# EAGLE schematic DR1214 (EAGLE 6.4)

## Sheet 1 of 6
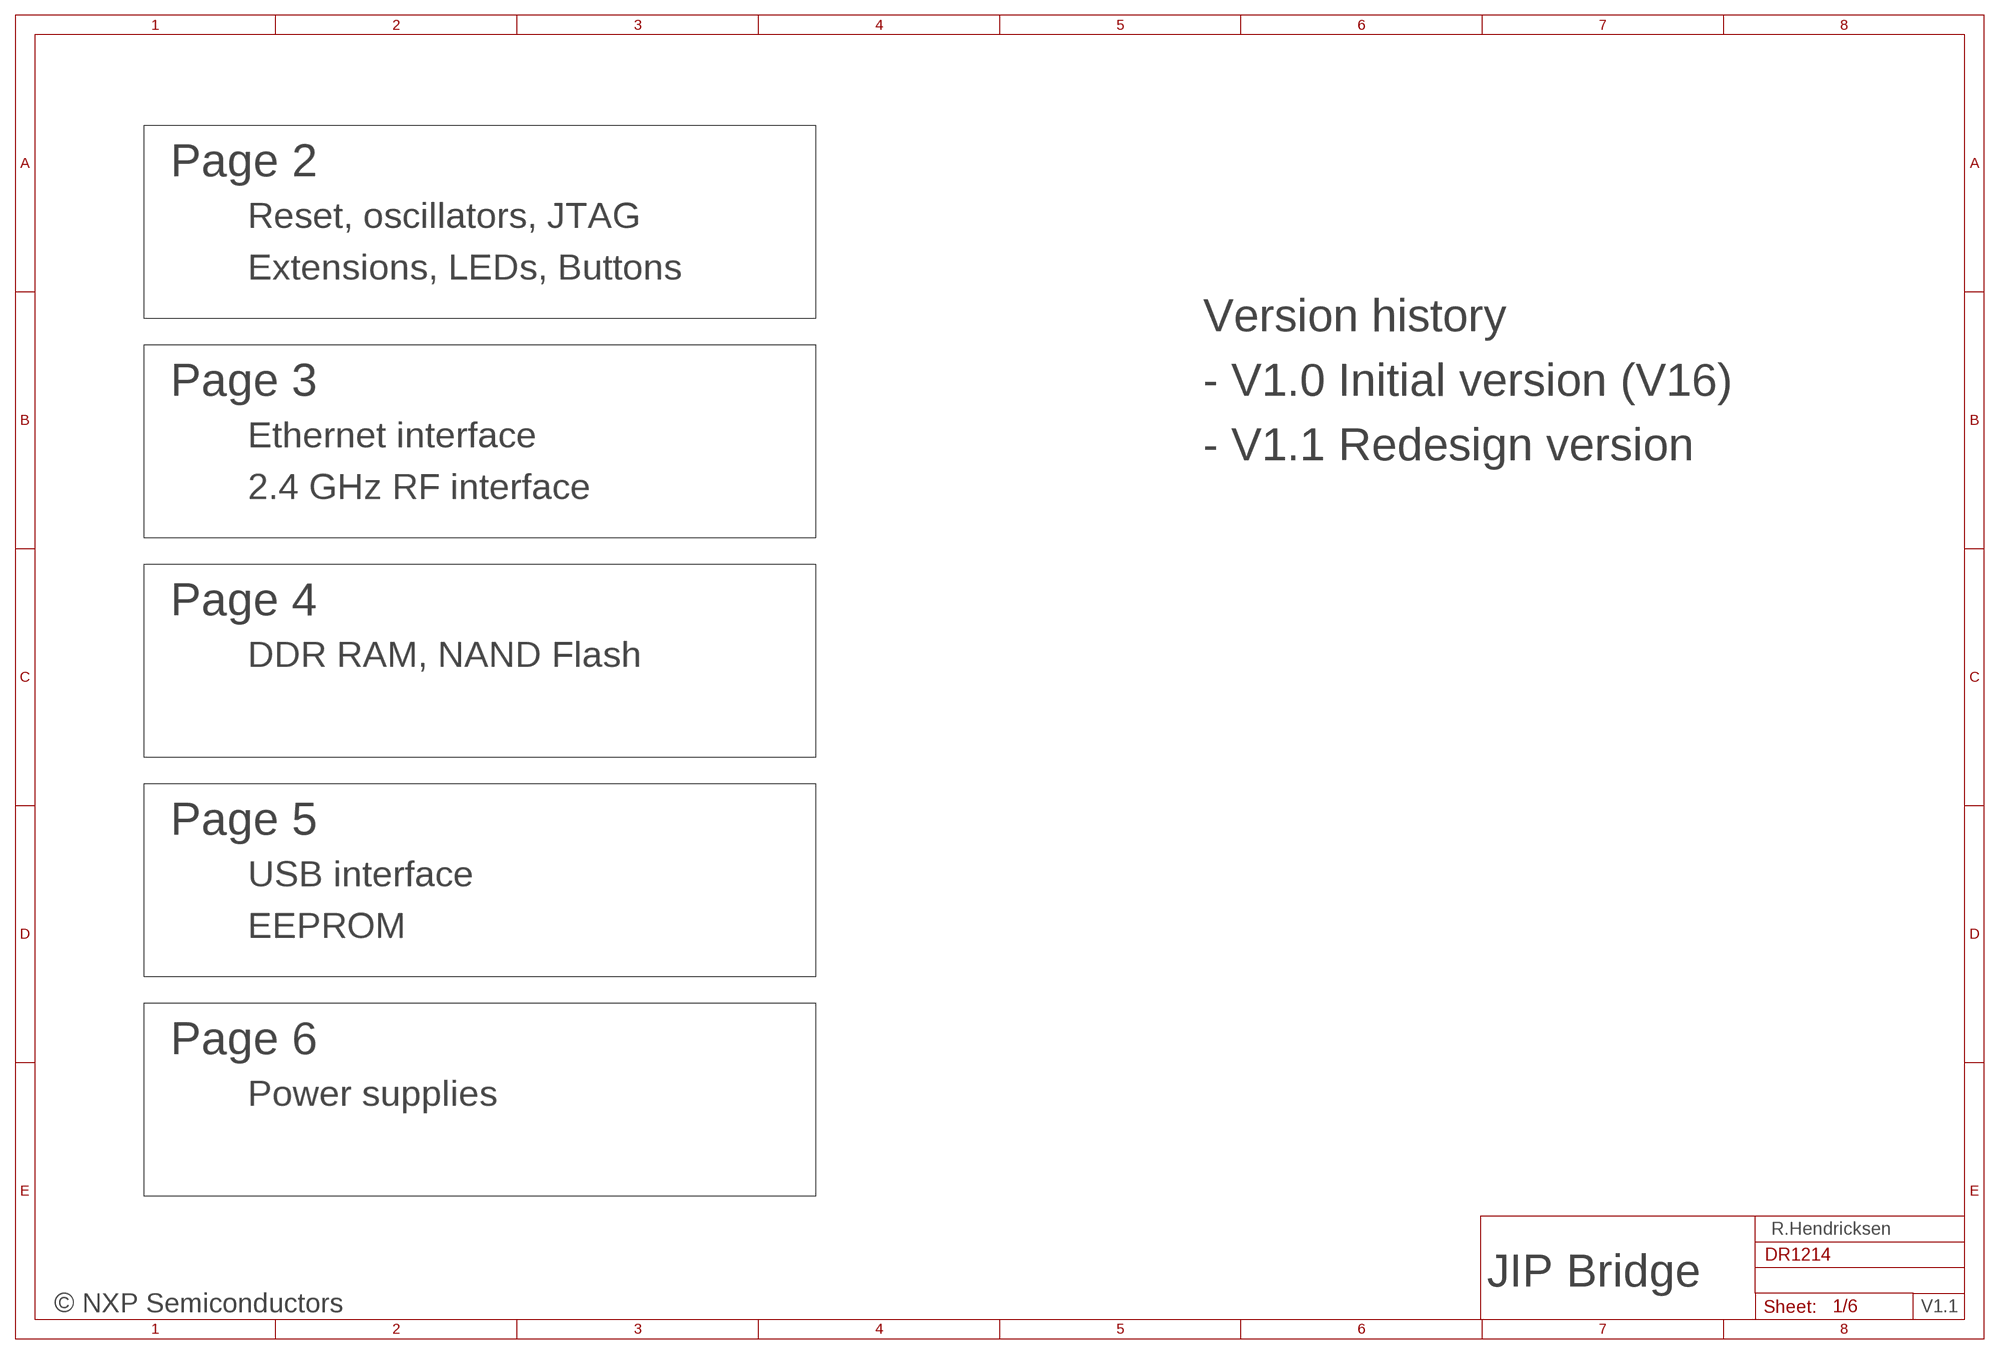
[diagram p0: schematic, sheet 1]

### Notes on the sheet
- Page 2
- Reset, oscillators, JTAG
- Extensions, LEDs, Buttons
- Version history
- Page 3 | - V1.0 Initial version (V16)
- Ethernet interface
- - V1.1 Redesign version
- 2.4 GHz RF interface
- Page 4
- DDR RAM, NAND Flash
- Page 5
- USB interface
- EEPROM
- Page 6
- Power supplies
- R.Hendricksen
- JIP Bridge
- © NXP Semiconductors | V1.1

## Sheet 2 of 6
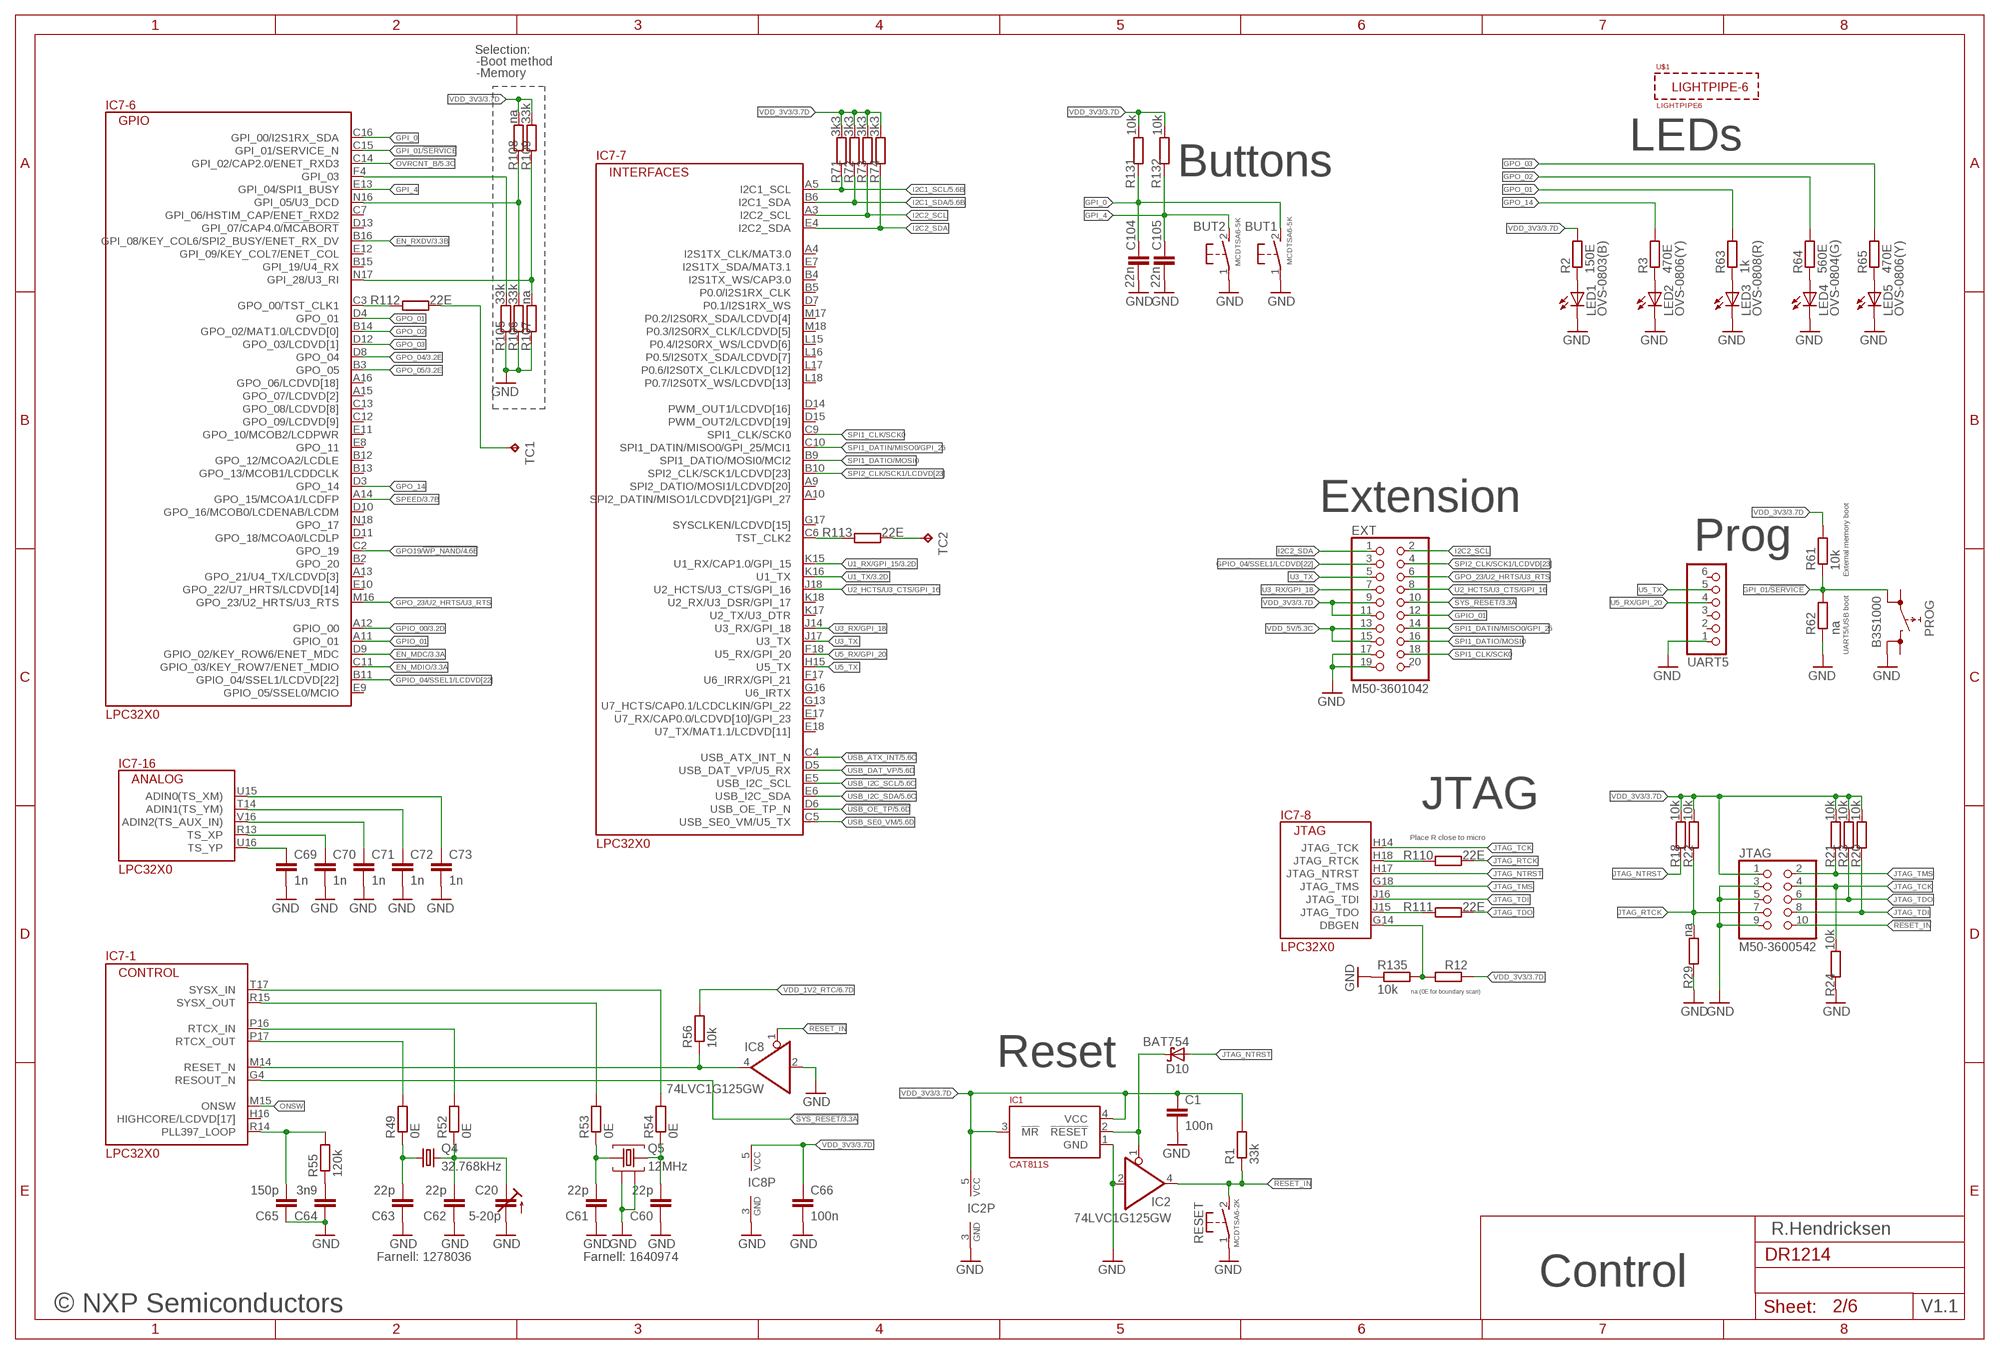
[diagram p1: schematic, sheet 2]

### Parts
BUT1  MCDTSA6-5K  MCDTSA6  [TACT90L]
BUT2  MCDTSA6-5K  MCDTSA6  [TACT90L]
C1  100n  C-EUC0402  [C0402]
C20  5-20p  C-TRIMMCTZ3  [CTRIMCTZ3]
C60  22p  C-EUC0402  [C0402]
C61  22p  C-EUC0402  [C0402]
C62  22p  C-EUC0402  [C0402]
C63  22p  C-EUC0402  [C0402]
C64  3n9  C-EUC0402  [C0402]
C65  150p  C-EUC0402  [C0402]
C66  100n  C-EUC0402  [C0402]
C69  1n  C-EUC0402  [C0402]
C70  1n  C-EUC0402  [C0402]
C71  1n  C-EUC0402  [C0402]
C72  1n  C-EUC0402  [C0402]
C73  1n  C-EUC0402  [C0402]
C104  22n  C-EUC0402  [C0402]
C105  22n  C-EUC0402  [C0402]
D10  BAT754  BAS16  [SOT23]
EXT  M50-3601042  [127_2R20_SMT]
IC1  CAT811S  [SOT143]
IC2  74LVC1G125GW  74LVC1G125DCK  [SC70-5]
IC7  LPC32X0  [SOT1048-1]
IC8  74LVC1G125GW  74LVC1G125DCK  [SC70-5]
JTAG  M50-3600542  [127_2R10_SMT]
LED1  OVS-0803(B)  [CHIPLED_0805]
LED2  OVS-0806(Y)  [CHIPLED_0805]
LED3  OVS-0808(R)  [CHIPLED_0805]
LED4  OVS-0804(G)  [CHIPLED_0805]
LED5  OVS-0806(Y)  [CHIPLED_0805]
PROG  B3S1000  [B3XS]
Q4  32.768kHz  RTCCRYSTAL  [XTAL2]
Q5  12MHz  CRYSTAL4  [XTAL4]
R1  33k  R-EU_R0402  [R0402]
R2  150E  R-EU_R0402  [R0402]
R3  470E  R-EU_R0402  [R0402]
R12  na (0E for boundary scan)  R-EU_R0402  [R0402]
R18  10k  R-EU_R0402  [R0402]
R20  10k  R-EU_R0402  [R0402]
R21  10k  R-EU_R0402  [R0402]
R22  10k  R-EU_R0402  [R0402]
R23  10k  R-EU_R0402  [R0402]
R24  10k  R-EU_R0402  [R0402]
R29  na  R-EU_R0402  [R0402]
R49  0E  R-EU_R0402  [R0402]
R52  0E  R-EU_R0402  [R0402]
R53  0E  R-EU_R0402  [R0402]
R54  0E  R-EU_R0402  [R0402]
R55  120k  R-EU_R0402  [R0402]
R56  10k  R-EU_R0402  [R0402]
R61  10k  R-EU_R0402  [R0402]
R62  na  R-EU_R0402  [R0402]
R63  1k  R-EU_R0402  [R0402]
R64  560E  R-EU_R0402  [R0402]
R65  470E  R-EU_R0402  [R0402]
R71  3k3  R-EU_R0402  [R0402]
R72  3k3  R-EU_R0402  [R0402]
R73  3k3  R-EU_R0402  [R0402]
R74  3k3  R-EU_R0402  [R0402]
R105  33k  R-EU_R0402  [R0402]
R106  33k  R-EU_R0402  [R0402]
R107  na  R-EU_R0402  [R0402]
R108  na  R-EU_R0402  [R0402]
R109  33k  R-EU_R0402  [R0402]
R110  22E  R-EU_R0402  [R0402]
R111  22E  R-EU_R0402  [R0402]
R112  22E  R-EU_R0402  [R0402]
R113  22E  R-EU_R0402  [R0402]
R131  10k  R-EU_R0402  [R0402]
R132  10k  R-EU_R0402  [R0402]
R135  10k  R-EU_R0402  [R0402]
RESET  MCDTSA6-2K  [TACT90]
TC1  TPB1,27  [B1,27]
TC2  TPB1,27  [B1,27]
U$1  LIGHTPIPE6  [LIGHTPIPE6]
UART5  PINHD-1X06_2.54-SMD  [1X06SMD]

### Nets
!RESET_IN: IC2.4(O) IC8.1(OE) JTAG.10 R1.1 RESET.2(S)
!SYS_RESET: EXT.10 IC7.G4(-1:RESOUT_N) ; also sheet 3,5
!USB_ATX_INT: IC7.C4(-7:USB_ATX_INT_N) ; also sheet 5
!USB_OE_TP: IC7.D6(-7:USB_OE_TP_N) ; also sheet 5
EN_MDC: IC7.D9(-6:GPIO_02/KEY_ROW6/ENET_MDC) ; also sheet 3
EN_MDIO: IC7.C11(-6:GPIO_03/KEY_ROW7/ENET_MDIO) ; also sheet 3
EN_RXDV: IC7.B16(-6:GPI_08/KEY_COL6/SPI2_BUSY/ENET_RX_DV) ; also sheet 3
GND [med_pow]: BUT1.1(P) BUT2.1(P) C1.2 C20.2(A) C60.1 C61.1 C62.1 C63.1 C64.1 C65.1 C66.2 C69.2 C70.2 C71.2 C72.2 C73.2 C104.2 C105.2 EXT.17 EXT.19 IC1.1(GND) IC2.2(I) IC2.3(GND) IC8.2(I) IC8.3(GND) JTAG.3 JTAG.5 JTAG.9 LED1.C LED2.C LED3.C LED4.C LED5.C PROG.4 Q5.2 Q5.4 R24.1 R29.1 R62.1 R105.1 R106.1 R107.1 R135.1 RESET.1(P) UART5.1 ; also sheet 3,4,5,6
GPI_0: BUT1.2(S) C104.1 IC7.C16(-6:GPI_00/I2S1RX_SDA) R131.1
GPI_01/!SERVICE: IC7.C15(-6:GPI_01/SERVICE_N) PROG.2 R61.1 R62.2
GPI_4: BUT2.2(S) C105.1 IC7.E13(-6:GPI_04/SPI1_BUSY) R132.1
GPIO_00: IC7.A12(-6:GPIO_00) ; also sheet 3
GPIO_01: EXT.12 IC7.A11(-6:GPIO_01)
GPIO_04/SSEL1/LCDVD[22]: EXT.3 IC7.B11(-6:GPIO_04/SSEL1/LCDVD[22])
GPO19/!WP_NAND: IC7.C2(-6:GPO_19) ; also sheet 4
GPO_01: IC7.D4(-6:GPO_01) R63.2
GPO_02: IC7.B14(-6:GPO_02/MAT1.0/LCDVD[0]) R64.2
GPO_03: IC7.D12(-6:GPO_03/LCDVD[1]) R65.2
GPO_04: IC7.D8(-6:GPO_04) ; also sheet 3
GPO_05: IC7.B3(-6:GPO_05) ; also sheet 3
GPO_14: IC7.D3(-6:GPO_14) R3.2
GPO_23/U2_HRTS/U3_RTS: EXT.6 IC7.M16(-6:GPO_23/U2_HRTS/U3_RTS)
I2C1_SCL: IC7.A5(-7:I2C1_SCL) R71.1 ; also sheet 5
I2C1_SDA: IC7.B6(-7:I2C1_SDA) R72.1 ; also sheet 5
I2C2_SCL: EXT.2 IC7.A3(-7:I2C2_SCL) R73.1
I2C2_SDA: EXT.1 IC7.E4(-7:I2C2_SDA) R74.1
JTAG_NTRST: D10.1(A) IC7.H17(-8:JTAG_NTRST) R18.1
JTAG_RTCK: JTAG.7 R22.1 R29.2 R110.2
JTAG_TCK: IC7.H14(-8:JTAG_TCK) JTAG.4 R24.2
JTAG_TDI: IC7.J16(-8:JTAG_TDI) JTAG.8 R20.1
JTAG_TDO: JTAG.6 R23.1 R111.2
JTAG_TMS: IC7.G18(-8:JTAG_TMS) JTAG.2 R21.1
N$2: D10.3(C) IC1.2(!RESET) IC2.1(OE)
N$3: LED1.A R2.1
N$4: LED2.A R3.1
N$18: C65.2 IC7.R14(-1:PLL397_LOOP) R55.2
N$23: IC7.G14(-8:DBGEN) R12.2 R135.2
N$25: C63.2 Q4.1 R49.1
N$26: C61.2 Q5.1 R53.1
N$30: C60.2 Q5.3 R54.1
N$34: C20.1(E) C62.2 Q4.2 R52.1
N$35: IC7.P17(-1:RTCX_OUT) R49.2
N$38: IC7.P16(-1:RTCX_IN) R52.2
N$41: IC7.R15(-1:SYSX_OUT) R53.2
N$42: IC7.T17(-1:SYSX_IN) R54.2
N$43: C64.2 R55.1
N$45: IC7.M14(-1:RESET_N) IC8.4(O) R56.1
N$46: LED3.A R63.1
N$50: LED4.A R64.1
N$52: LED5.A R65.1
N$73: C69.1 IC7.U16(-16:TS_YP)
N$74: C70.1 IC7.R13(-16:TS_XP)
N$75: C71.1 IC7.V16(-16:ADIN2(TS_AUX_IN))
N$76: C72.1 IC7.T14(-16:ADIN1(TS_YM))
N$77: C73.1 IC7.U15(-16:ADIN0(TS_XM))
N$138: IC7.F4(-6:GPI_03) R105.2
N$140: IC7.N16(-6:GPI_05/U3_DCD) R106.2 R108.1
N$141: IC7.N17(-6:GPI_28/U3_RI) R107.2 R109.1
N$142: IC7.H18(-8:JTAG_RTCK) R110.1
N$143: IC7.J15(-8:JTAG_TDO) R111.1
N$144: IC7.C3(-6:GPO_00/TST_CLK1) R112.1
N$146: IC7.C6(-7:TST_CLK2) R113.1
ONSW: IC7.M15(-1:ONSW)
OVRCNT_B: IC7.C14(-6:GPI_02/CAP2.0/ENET_RXD3) ; also sheet 5
SPEED: IC7.A14(-6:GPO_15/MCOA1/LCDFP) ; also sheet 3
SPI1_CLK/SCK0: EXT.18 IC7.C9(-7:SPI1_CLK/SCK0)
SPI1_DATIN/MISO0/GPI_25: EXT.14 IC7.C10(-7:SPI1_DATIN/MISO0/GPI_25/MCI1)
SPI1_DATIO/MOSI0: EXT.16 IC7.B9(-7:SPI1_DATIO/MOSI0/MCI2)
SPI2_CLK/SCK1/LCDVD[23]: EXT.4 IC7.B10(-7:SPI2_CLK/SCK1/LCDVD[23])
TC1: R112.2 TC1.TP
TC2: R113.2 TC2.TP
U1_RX/GPI_15: IC7.K15(-7:U1_RX/CAP1.0/GPI_15) ; also sheet 3
U1_TX: IC7.K16(-7:U1_TX) ; also sheet 3
U2_HCTS/U3_CTS/GPI_16: EXT.8 IC7.J18(-7:U2_HCTS/U3_CTS/GPI_16)
U3_RX/GPI_18: EXT.7 IC7.J14(-7:U3_RX/GPI_18)
U3_TX: EXT.5 IC7.J17(-7:U3_TX)
U5_RX/GPI_20: IC7.F18(-7:U5_RX/GPI_20) UART5.4
U5_TX: IC7.H15(-7:U5_TX) UART5.5
USB_DAT_VP: IC7.D5(-7:USB_DAT_VP/U5_RX) ; also sheet 5
USB_I2C_SCL: IC7.E5(-7:USB_I2C_SCL) ; also sheet 5
USB_I2C_SDA: IC7.E6(-7:USB_I2C_SDA) ; also sheet 5
USB_SE0_VM: IC7.C5(-7:USB_SE0_VM/U5_TX) ; also sheet 5
VDD_1V2_RTC: R56.2 ; also sheet 6
VDD_3V3: C1.1 C66.1 EXT.9 EXT.11 IC1.3(!MR) IC1.4(VCC) IC2.5(VCC) IC8.5(VCC) JTAG.1 R1.2 R2.2 R12.1 R18.2 R20.2 R21.2 R22.2 R23.2 R61.2 R71.2 R72.2 R73.2 R74.2 R108.2 R109.2 R131.2 R132.2 ; also sheet 3,4,5,6
VDD_5V: EXT.13 EXT.15 ; also sheet 5,6
Unconnected: EXT.20 IC7.A4(-7:I2S1TX_CLK/MAT3.0) IC7.A9(-7:SPI2_DATIO/MOSI1/LCDVD[20]) IC7.A10(-7:SPI2_DATIN/MISO1/LCDVD[21]/GPI_27) IC7.A13(-6:GPO_21/U4_TX/LCDVD[3]) IC7.A15(-6:GPO_07/LCDVD[2]) IC7.A16(-6:GPO_06/LCDVD[18]) IC7.B2(-6:GPO_20) IC7.B4(-7:I2S1TX_WS/CAP3.0) IC7.B5(-7:P0.0/I2S1RX_CLK) IC7.B12(-6:GPO_12/MCOA2/LCDLE) IC7.B13(-6:GPO_13/MCOB1/LCDDCLK) IC7.B15(-6:GPI_19/U4_RX) IC7.C7(-6:GPI_06/HSTIM_CAP/ENET_RXD2) IC7.C12(-6:GPO_09/LCDVD[9]) IC7.C13(-6:GPO_08/LCDVD[8]) IC7.D7(-7:P0.1/I2S1RX_WS) IC7.D10(-6:GPO_16/MCOB0/LCDENAB/LCDM) IC7.D11(-6:GPO_18/MCOA0/LCDLP) IC7.D13(-6:GPI_07/CAP4.0/!MCABORT) IC7.D14(-7:PWM_OUT1/LCDVD[16]) IC7.D15(-7:PWM_OUT2/LCDVD[19]) IC7.E7(-7:I2S1TX_SDA/MAT3.1) IC7.E8(-6:GPO_11) IC7.E9(-6:GPIO_05/SSEL0/MCIO) IC7.E10(-6:GPO_22/U7_HRTS/LCDVD[14]) IC7.E11(-6:GPO_10/MCOB2/LCDPWR) IC7.E12(-6:GPI_09/KEY_COL7/ENET_COL) IC7.E17(-7:U7_RX/CAP0.0/LCDVD[10]/GPI_23) IC7.E18(-7:U7_TX/MAT1.1/LCDVD[11]) IC7.F17(-7:U6_IRRX/GPI_21) IC7.G13(-7:U7_HCTS/CAP0.1/LCDCLKIN/GPI_22) IC7.G16(-7:U6_IRTX) IC7.G17(-7:SYSCLKEN/LCDVD[15]) IC7.H16(-1:HIGHCORE/LCDVD[17]) IC7.K17(-7:U2_TX/U3_DTR) IC7.K18(-7:U2_RX/U3_DSR/GPI_17) IC7.L15(-7:P0.4/I2S0RX_WS/LCDVD[6]) IC7.L16(-7:P0.5/I2S0TX_SDA/LCDVD[7]) IC7.L17(-7:P0.6/I2S0TX_CLK/LCDVD[12]) IC7.L18(-7:P0.7/I2S0TX_WS/LCDVD[13]) IC7.M17(-7:P0.2/I2S0RX_SDA/LCDVD[4]) IC7.M18(-7:P0.3/I2S0RX_CLK/LCDVD[5]) IC7.N18(-6:GPO_17) PROG.1 PROG.3 UART5.2 UART5.3 UART5.6

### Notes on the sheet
- Selection:
- -Boot method
- -Memory
- LEDs
- Buttons
- Extension
- Prog
- External memory boot
- UART5/USB boot
- JTAG
- Place R close to micro
- Reset
- R.Hendricksen
- Farnell: 1278036 | Farnell: 1640974
- Control
- © NXP Semiconductors | V1.1

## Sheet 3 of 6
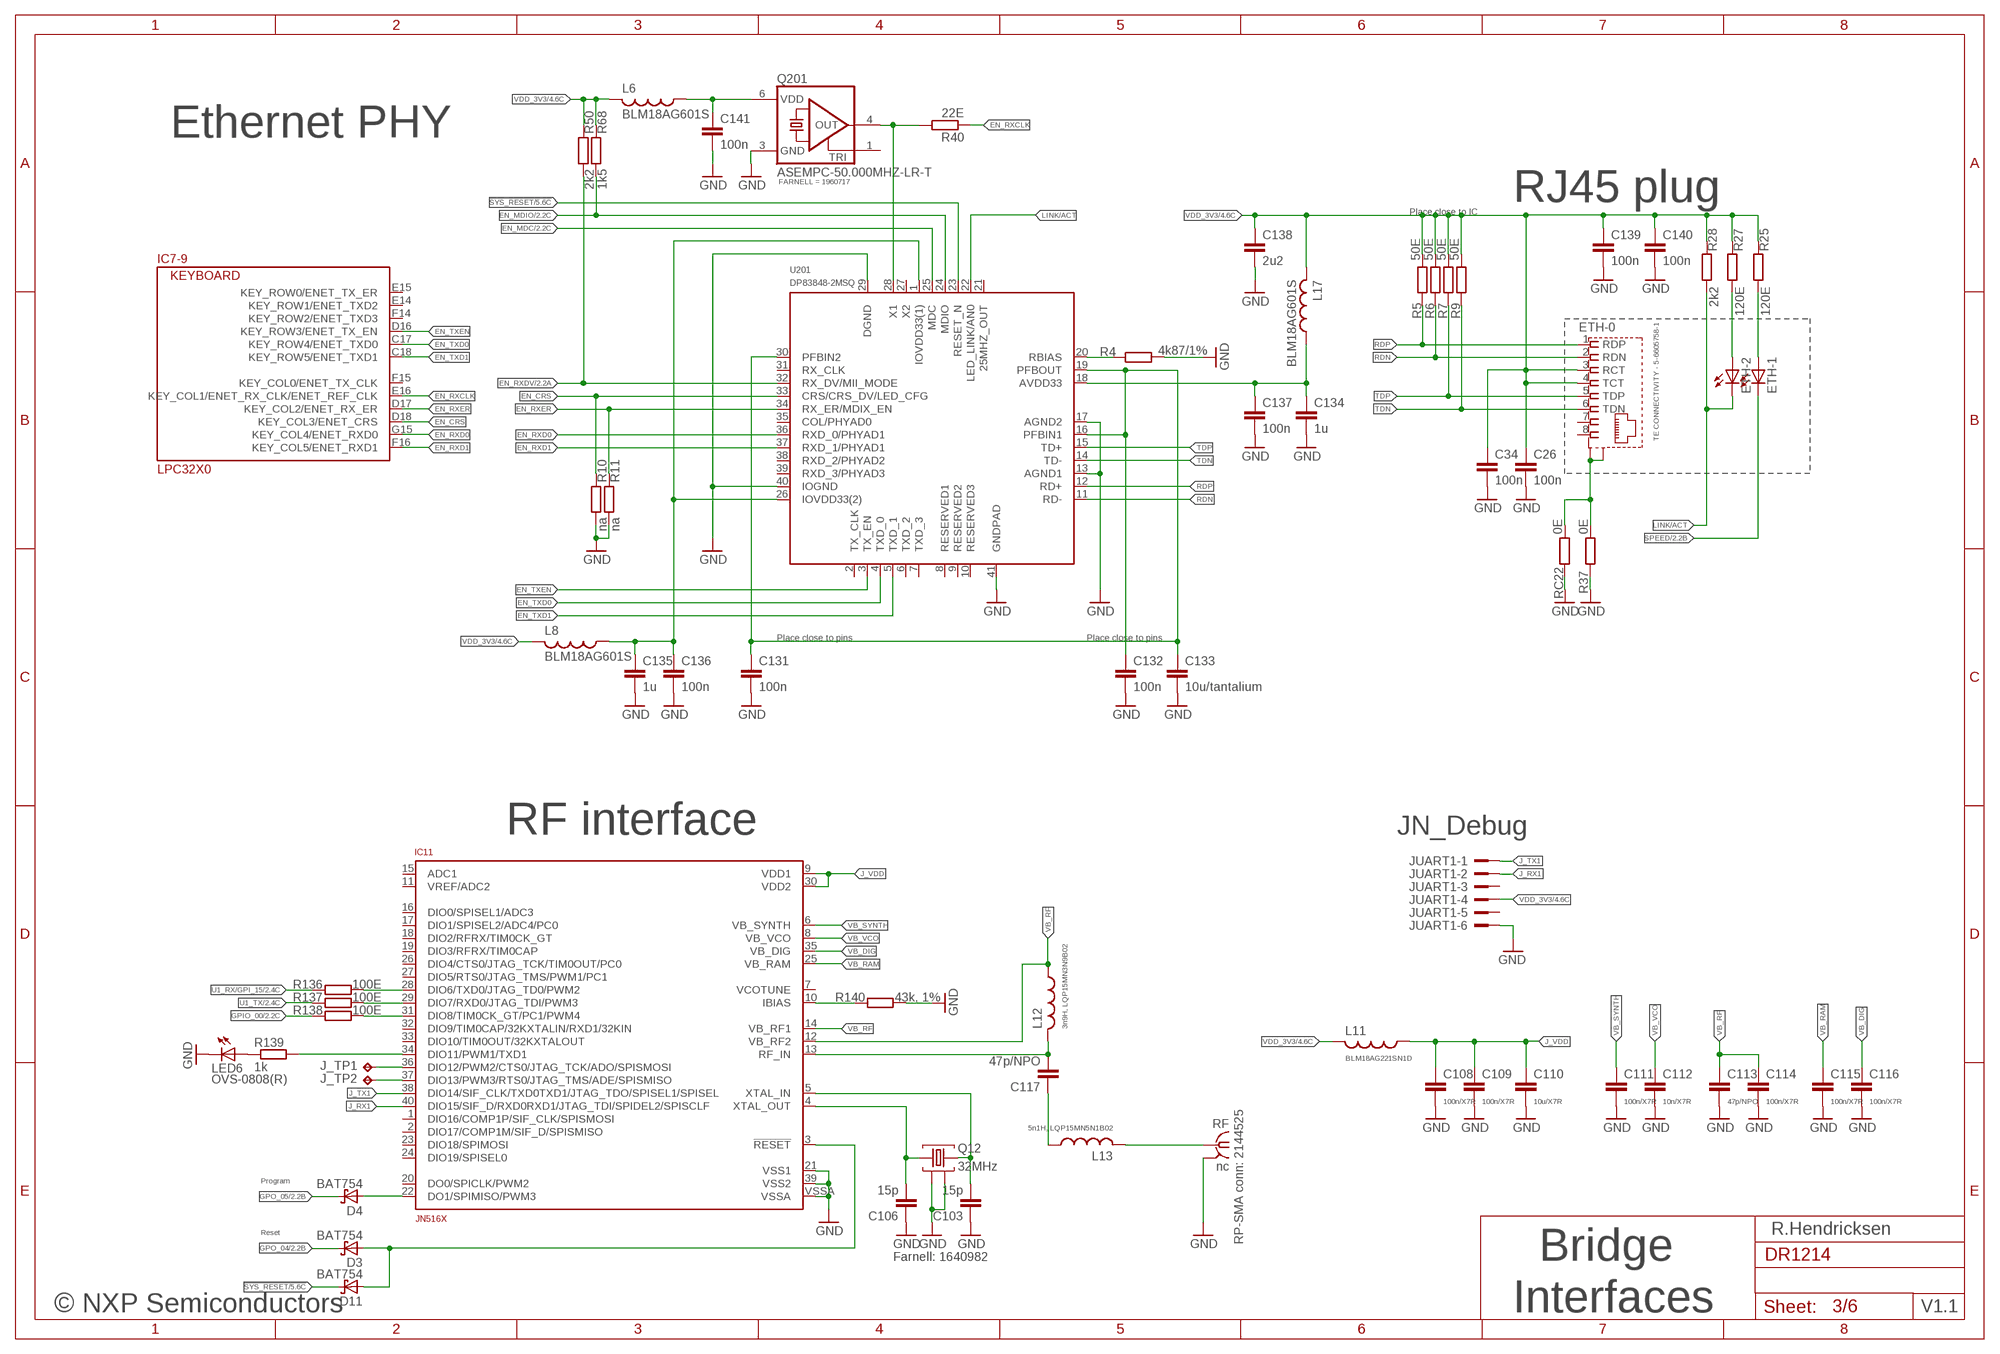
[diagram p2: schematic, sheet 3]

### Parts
C26  100n  C-EUC0402  [C0402]
C34  100n  C-EUC0402  [C0402]
C103  15p  C-EUC0402  [C0402]
C106  15p  C-EUC0402  [C0402]
C108  100n/X7R  C-EUC0402  [C0402]
C109  100n/X7R  C-EUC0402  [C0402]
C110  10u/X7R  C-EUC0805  [C0805]
C111  100n/X7R  C-EUC0402  [C0402]
C112  10n/X7R  C-EUC0402  [C0402]
C113  47p/NPO  C-EUC0402  [C0402]
C114  100n/X7R  C-EUC0402  [C0402]
C115  100n/X7R  C-EUC0402  [C0402]
C116  100n/X7R  C-EUC0402  [C0402]
C117  47p/NPO  C-EUC0402  [C0402]
C131  100n  C-EUC0402  [C0402]
C132  100n  C-EUC0402  [C0402]
C133  10u/tantalium  C-EUC1206  [C1206]
C134  1u  C-EUC0402  [C0402]
C135  1u  C-EUC0402  [C0402]
C136  100n  C-EUC0402  [C0402]
C137  100n  C-EUC0402  [C0402]
C138  2u2  C-EUC0402  [C0402]
C139  100n  C-EUC0402  [C0402]
C140  100n  C-EUC0402  [C0402]
C141  100n  C-EUC0402  [C0402]
D3  BAT754  BAS16  [SOT23]
D4  BAT754  BAS16  [SOT23]
D11  BAT754  BAS16  [SOT23]
ETH  TE CONNECTIVITY - 5-6605758-1  JACK8LED_RH  [MODULARJACK8_L]
IC11  JN516X  [SOT618-1]
J_TP1  TPB1,27  [B1,27]
J_TP2  TPB1,27  [B1,27]
JUART1  BD075-06-A-1-L-D  [BD075-06-A-1-L-D]
L6  BLM18AG601S  [PACKAGE0603]
L8  BLM18AG601S  [PACKAGE0603]
L11  BLM18AG221SN1D  L_0603  [R0603]
L12  3n9H, LQP15MN3N9B02  L0603  [P0603]
L13  5n1H, LQP15MN5N1B02  L0603  [P0603]
L17  BLM18AG601S  [PACKAGE0603]
LED6  OVS-0808(R)  [CHIPLED_0805]
Q12  32MHz  CRYSTAL4  [XTAL4]
Q201  ASEMPC-50.000MHZ-LR-T  [ASE]
R4  4k87/1%  R-EU_R0402  [R0402]
R5  50E  R-EU_R0402  [R0402]
R6  50E  R-EU_R0402  [R0402]
R7  50E  R-EU_R0402  [R0402]
R9  50E  R-EU_R0402  [R0402]
R10  na  R-EU_R0402  [R0402]
R11  na  R-EU_R0402  [R0402]
R25  120E  R-EU_R0402  [R0402]
R27  120E  R-EU_R0402  [R0402]
R28  2k2  R-EU_R0402  [R0402]
R37  0E  R-EU_R1206  [R1206]
R40  22E  R-EU_R0402  [R0402]
R50  2k2  R-EU_R0402  [R0402]
R68  1k5  R-EU_R0402  [R0402]
R136  100E  R-EU_R0402  [R0402]
R137  100E  R-EU_R0402  [R0402]
R138  100E  R-EU_R0402  [R0402]
R139  1k  R-EU_R0402  [R0402]
R140  43k, 1%  R-EU_R0402  [R0402]
RC22  0E  R-EU_R1206  [R1206]
RF  nc  BU-SMA-V  [BU-SMA-V]
U201  DP83848-2MSQ  [MVER_ETHERNET_LLP40]

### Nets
!SYS_RESET: D11.3(C) U201.23(RESET_N) ; also sheet 2,5
EN_CRS: IC7.D18(-9:KEY_COL3/ENET_CRS) R10.1 U201.33(CRS/CRS_DV/LED_CFG)
EN_MDC: U201.25(MDC) ; also sheet 2
EN_MDIO: R68.2 U201.24(MDIO) ; also sheet 2
EN_RXCLK: IC7.E16(-9:KEY_COL1/ENET_RX_CLK/ENET_REF_CLK) R40.1
EN_RXD0: IC7.G15(-9:KEY_COL4/ENET_RXD0) U201.36(RXD_0/PHYAD1)
EN_RXD1: IC7.F16(-9:KEY_COL5/ENET_RXD1) U201.37(RXD_1/PHYAD1)
EN_RXDV: R50.2 U201.32(RX_DV/MII_MODE) ; also sheet 2
EN_RXER: IC7.D17(-9:KEY_COL2/ENET_RX_ER) R11.1 U201.34(RX_ER/MDIX_EN)
EN_TXD0: IC7.C17(-9:KEY_ROW4/ENET_TXD0) U201.4(TXD_0)
EN_TXD1: IC7.C18(-9:KEY_ROW5/ENET_TXD1) U201.5(TXD_1)
EN_TXEN: IC7.D16(-9:KEY_ROW3/ENET_TX_EN) U201.3(TX_EN)
ETH_SHIELD: ETH.S1(-0:S1) ETH.S2(-0:S2) R37.2 RC22.1
GND [med_pow]: C26.2 C34.2 C103.1 C106.1 C108.2 C109.2 C110.2 C111.2 C112.2 C113.2 C114.2 C115.2 C116.2 C131.2 C132.2 C133.2 C134.2 C135.2 C136.2 C137.2 C138.2 C139.2 C140.2 C141.2 IC11.21(VSS1) IC11.39(VSS2) IC11.VSSA JUART1.6 LED6.C Q12.2 Q12.4 Q201.3(GND) R4.2 R10.2 R11.2 R37.1 R140.2 RC22.2 RF.2(GND) U201.13(AGND1) U201.17(AGND2) U201.29(DGND) U201.40(IOGND) U201.41(GNDPAD) ; also sheet 2,4,5,6
GPIO_00: R138.1 ; also sheet 2
GPO_04: D3.3(C) ; also sheet 2
GPO_05: D4.3(C) ; also sheet 2
J_RX1: IC11.40(DIO15/SIF_D/RXD0RXD1/JTAG_TDI/SPIDEL2/SPISCLF) JUART1.2
J_TX1: IC11.38(DIO14/SIF_CLK/TXD0TXD1/JTAG_TDO/SPISEL1/SPISEL) JUART1.1
J_VDD: C108.1 C109.1 C110.1 IC11.9(VDD1) IC11.30(VDD2) L11.1
LINK/ACT: ETH.C2(-2:C) R28.2 U201.22(LED_LINK/AN0)
N$1: Q201.4(OUT) R40.2 U201.28(X1)
N$6: R4.1 U201.20(RBIAS)
N$12: L13.2 RF.1
N$20: C134.1 C137.1 L17.1 U201.18(AVDD33)
N$31: ETH.A1(-1:A) R25.2
N$32: C141.1 L6.1 Q201.6(VDD)
N$39: ETH.A2(-2:A) R27.2
N$54: IC11.10(IBIAS) R140.1
N$55: C106.2 IC11.4(XTAL_OUT) Q12.1
N$159: IC11.29(DIO7/RXD0/JTAG_TDI/PWM3) R137.2
N$160: IC11.31(DIO8/TIM0CK_GT/PC1/PWM4) R138.2
N$161: D3.1(A) D11.1(A) IC11.3(!RESET)
N$162: IC11.28(DIO6/TXD0/JTAG_TD0/PWM2) R136.2
N$163: D4.1(A) IC11.22(DO1/SPIMISO/PWM3)
N$164: LED6.A R139.1
N$165: IC11.34(DIO11/PWM1/TXD1) R139.2
N$166: IC11.37(DIO13/PWM3/RTS0/JTAG_TMS/ADE/SPISMISO) J_TP2.TP
N$167: IC11.36(DIO12/PWM2/CTS0/JTAG_TCK/ADO/SPISMOSI) J_TP1.TP
N$168: C103.2 IC11.5(XTAL_IN) Q12.3
N$169: C117.2 IC11.13(RF_IN) L12.2
N$170: C117.1 L13.1
RDN: ETH.2(-0:RDN) R6.1 U201.11(RD-)
RDP: ETH.1(-0:RDP) R5.1 U201.12(RD+)
RFBOUT: C131.1 C132.1 C133.1 U201.16(PFBIN1) U201.19(PFBOUT) U201.30(PFBIN2)
SPEED: ETH.C1(-1:C) ; also sheet 2
TDN: ETH.6(-0:TDN) R9.1 U201.14(TD-)
TDP: ETH.5(-0:TDP) R7.1 U201.15(TD+)
U1_RX/GPI_15: R136.1 ; also sheet 2
U1_TX: R137.1 ; also sheet 2
VB_DIG: C116.1 IC11.35(VB_DIG)
VB_RAM: C115.1 IC11.25(VB_RAM)
VB_RF: C113.1 C114.1 IC11.12(VB_RF2) IC11.14(VB_RF1) L12.1
VB_SYNTH: C111.1 IC11.6(VB_SYNTH)
VB_VCO: C112.1 IC11.8(VB_VCO)
VDD_3V3: C26.1 C34.1 C138.1 C139.1 C140.1 ETH.3(-0:RCT) ETH.4(-0:TCT) JUART1.4 L6.2 L8.2 L11.2 L17.2 R5.2 R6.2 R7.2 R9.2 R25.1 R27.1 R28.1 R50.1 R68.1 ; also sheet 2,4,5,6
VDD_ETH: C135.1 C136.1 L8.1 U201.1(IOVDD33(1)) U201.26(IOVDD33(2))
Unconnected: ETH.7 ETH.8 IC7.E14(-9:KEY_ROW1/ENET_TXD2) IC7.E15(-9:KEY_ROW0/ENET_TX_ER) IC7.F14(-9:KEY_ROW2/ENET_TXD3) IC7.F15(-9:KEY_COL0/ENET_TX_CLK) IC11.1(DIO16/COMP1P/SIF_CLK/SPISMOSI) IC11.2(DIO17/COMP1M/SIF_D/SPISMISO) IC11.7(VCOTUNE) IC11.11(VREF/ADC2) IC11.15(ADC1) IC11.16(DIO0/SPISEL1/ADC3) IC11.17(DIO1/SPISEL2/ADC4/PC0) IC11.18(DIO2/RFRX/TIM0CK_GT) IC11.19(DIO3/RFRX/TIM0CAP) IC11.20(DO0/SPICLK/PWM2) IC11.23(DIO18/SPIMOSI) IC11.24(DIO19/SPISEL0) IC11.26(DIO4/CTS0/JTAG_TCK/TIM0OUT/PC0) IC11.27(DIO5/RTS0/JTAG_TMS/PWM1/PC1) IC11.32(DIO9/TIM0CAP/32KXTALIN/RXD1/32KIN) IC11.33(DIO10/TIM0OUT/32KXTALOUT) JUART1.3 JUART1.5 Q201.1(TRI) U201.2(TX_CLK) U201.6(TXD_2) U201.7(TXD_3) U201.8(RESERVED1) U201.9(RESERVED2) U201.10(RESERVED3) U201.21(25MHZ_OUT) U201.27(X2) U201.31(RX_CLK) U201.35(COL/PHYAD0) U201.38(RXD_2/PHYAD2) U201.39(RXD_3/PHYAD3)

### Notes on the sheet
- Ethernet PHY
- RJ45 plug
- Place close to IC
- Place close to pins | Place close to pins
- RF interface | JN_Debug
- Program
- Reset | R.Hendricksen
- RP-SMA conn: 2144525
- Farnell: 1640982 | Bridge
- © NXP Semiconductors | Interfaces | V1.1

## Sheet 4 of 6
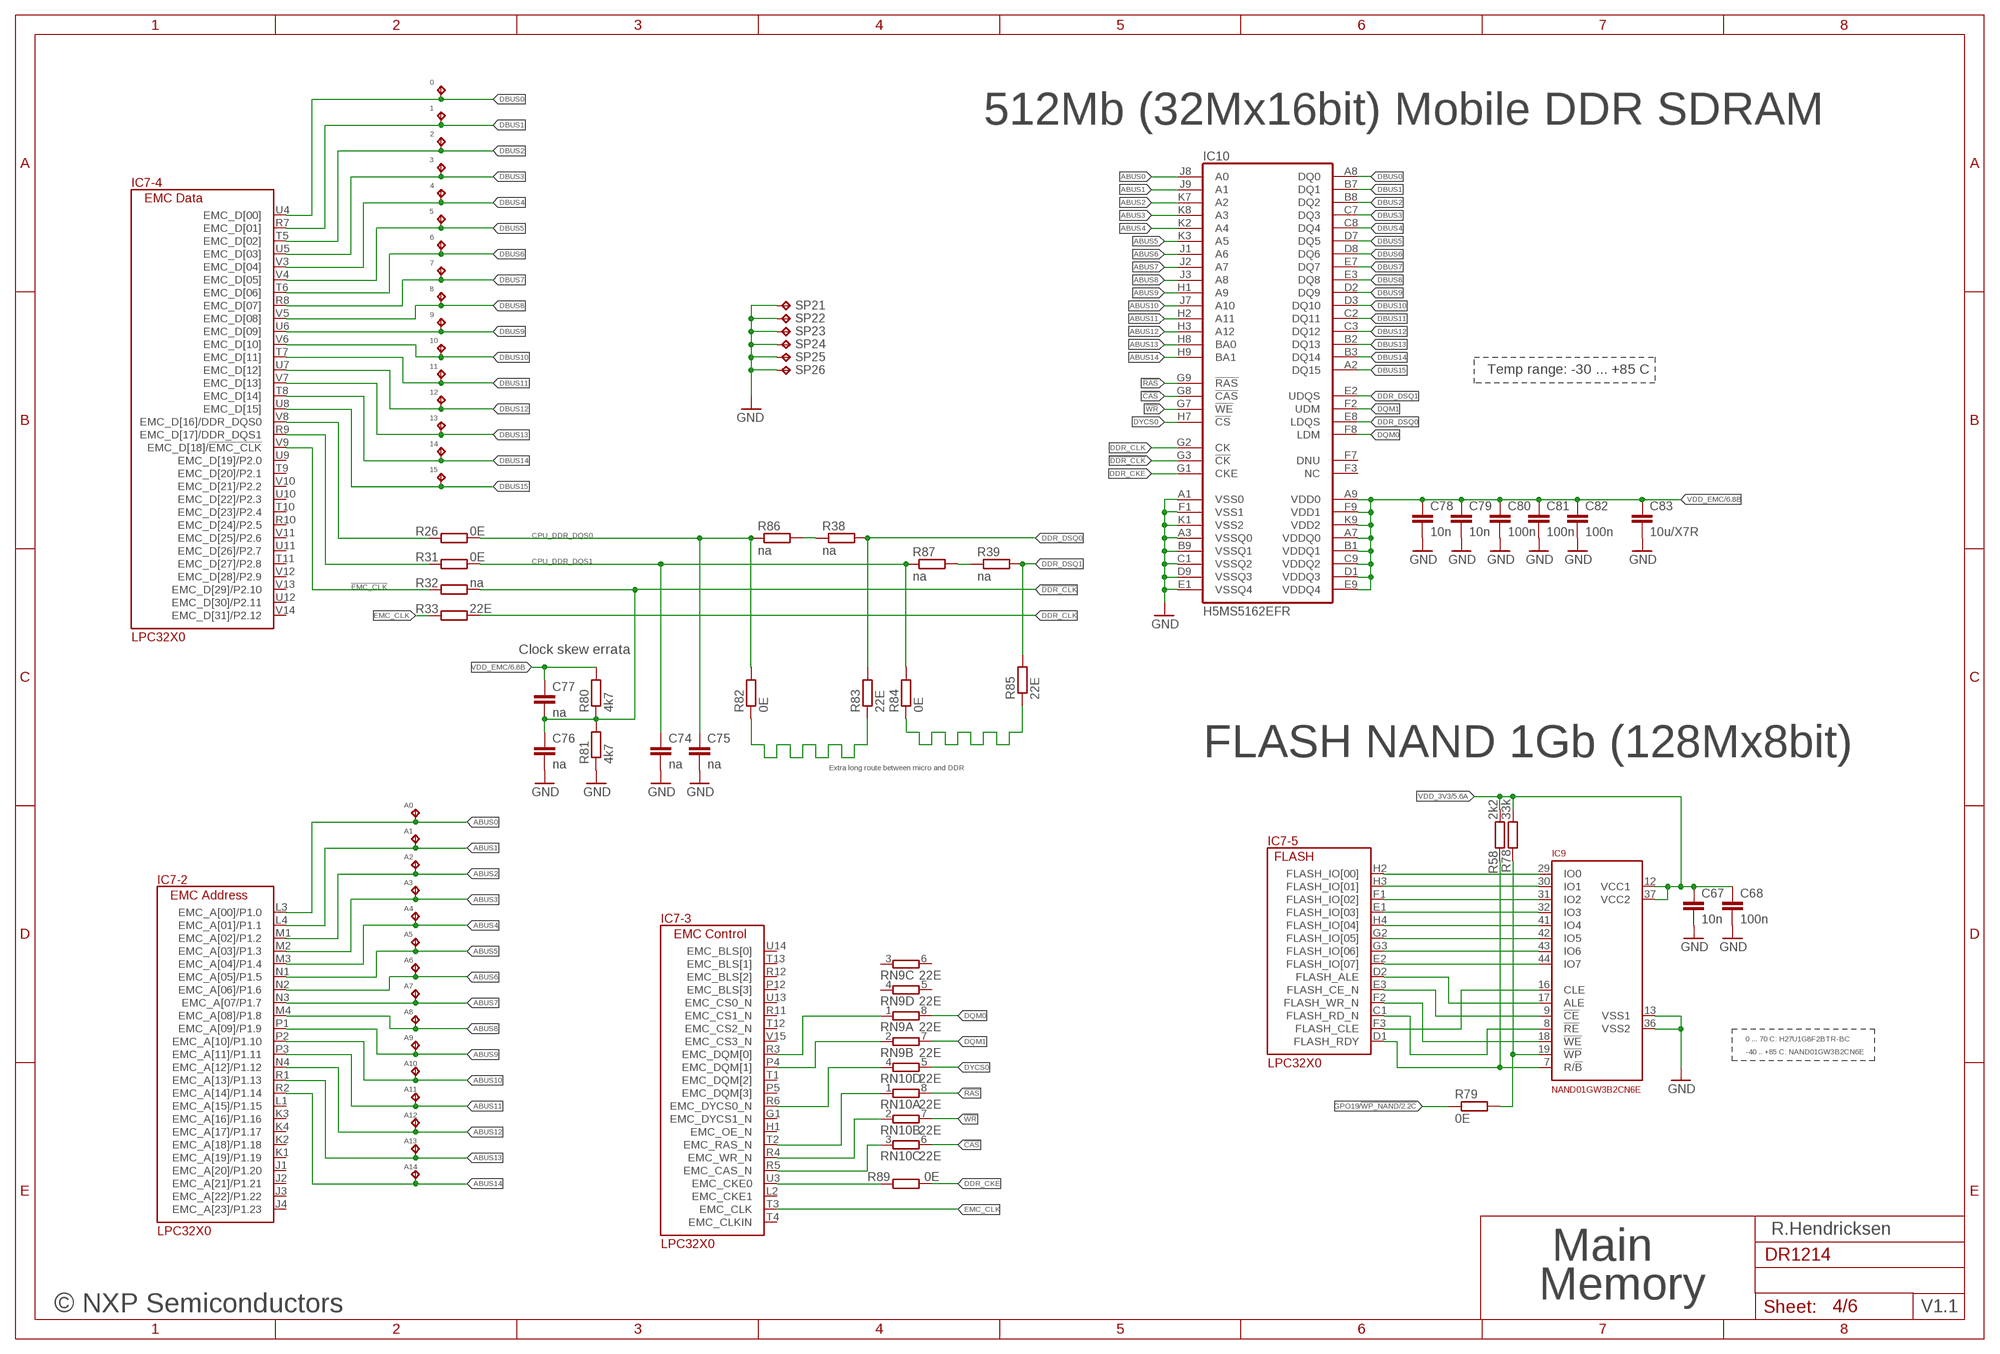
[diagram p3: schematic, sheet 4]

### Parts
0  TP0.5  [B0,5MM]
1  TP0.5  [B0,5MM]
2  TP0.5  [B0,5MM]
3  TP0.5  [B0,5MM]
4  TP0.5  [B0,5MM]
5  TP0.5  [B0,5MM]
6  TP0.5  [B0,5MM]
7  TP0.5  [B0,5MM]
8  TP0.5  [B0,5MM]
9  TP0.5  [B0,5MM]
10  TP0.5  [B0,5MM]
11  TP0.5  [B0,5MM]
12  TP0.5  [B0,5MM]
13  TP0.5  [B0,5MM]
14  TP0.5  [B0,5MM]
15  TP0.5  [B0,5MM]
A0  TP0.5  [B0,5MM]
A1  TP0.5  [B0,5MM]
A2  TP0.5  [B0,5MM]
A3  TP0.5  [B0,5MM]
A4  TP0.5  [B0,5MM]
A5  TP0.5  [B0,5MM]
A6  TP0.5  [B0,5MM]
A7  TP0.5  [B0,5MM]
A8  TP0.5  [B0,5MM]
A9  TP0.5  [B0,5MM]
A10  TP0.5  [B0,5MM]
A11  TP0.5  [B0,5MM]
A12  TP0.5  [B0,5MM]
A13  TP0.5  [B0,5MM]
A14  TP0.5  [B0,5MM]
C67  10n  C-EUC0402  [C0402]
C68  100n  C-EUC0402  [C0402]
C74  na  C-EUC0402  [C0402]
C75  na  C-EUC0402  [C0402]
C76  na  C-EUC0402  [C0402]
C77  na  C-EUC0402  [C0402]
C78  10n  C-EUC0402  [C0402]
C79  10n  C-EUC0402  [C0402]
C80  100n  C-EUC0402  [C0402]
C81  100n  C-EUC0402  [C0402]
C82  100n  C-EUC0402  [C0402]
C83  10u/X7R  C-EUC0805  [C0805]
IC9  NAND01GW3B2CN6E  H27U1G8F2BTR  [TSOP48]
IC10  H5MS5162EFR  [FBGA60-6X10]
R26  0E  R-EU_R0402  [R0402]
R31  0E  R-EU_R0402  [R0402]
R32  na  R-EU_R0402  [R0402]
R33  22E  R-EU_R0402  [R0402]
R38  na  R-EU_R0402  [R0402]
R39  na  R-EU_R0402  [R0402]
R58  2k2  R-EU_R0402  [R0402]
R78  33k  R-EU_R0402  [R0402]
R79  0E  R-EU_R0402  [R0402]
R80  4k7  R-EU_R0402  [R0402]
R81  4k7  R-EU_R0402  [R0402]
R82  0E  R-EU_R0402  [R0402]
R83  22E  R-EU_R0402  [R0402]
R84  0E  R-EU_R0402  [R0402]
R85  22E  R-EU_R0402  [R0402]
R86  na  R-EU_R0402  [R0402]
R87  na  R-EU_R0402  [R0402]
R89  0E  R-EU_R0402  [R0402]
RN9  22E  4R-NEXB18V  [EXB18V]
RN10  22E  4R-NEXB18V  [EXB18V]
SP21  TPTP06SQ  [TP06SQ]
SP22  TPTP06SQ  [TP06SQ]
SP23  TPTP06SQ  [TP06SQ]
SP24  TPTP06SQ  [TP06SQ]
SP25  TPTP06SQ  [TP06SQ]
SP26  TPTP06SQ  [TP06SQ]

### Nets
!CAS: IC10.G8(!CAS) RN10.6
!DDR_CLK: C76.1 C77.2 IC10.G3(!CK) R32.2 R80.1 R81.2
!EMC_CLK: IC7.V9(-4:EMC_D[18]/!EMC_CLK) R32.1
!RAS: IC10.G9(!RAS) RN10.8
!WR: IC10.G7(!WE) RN10.7
ABUS0: A0.TP IC7.L3(-2:EMC_A[00]/P1.0) IC10.J8(A0)
ABUS1: A1.TP IC7.L4(-2:EMC_A[01]/P1.1) IC10.J9(A1)
ABUS2: A2.TP IC7.M1(-2:EMC_A[02]/P1.2) IC10.K7(A2)
ABUS3: A3.TP IC7.M2(-2:EMC_A[03]/P1.3) IC10.K8(A3)
ABUS4: A4.TP IC7.M3(-2:EMC_A[04]/P1.4) IC10.K2(A4)
ABUS5: A5.TP IC7.N1(-2:EMC_A[05]/P1.5) IC10.K3(A5)
ABUS6: A6.TP IC7.N2(-2:EMC_A[06]/P1.6) IC10.J1(A6)
ABUS7: A7.TP IC7.N3(-2:EMC_A[07/P1.7) IC10.J2(A7)
ABUS8: A8.TP IC7.M4(-2:EMC_A[08]/P1.8) IC10.J3(A8)
ABUS9: A9.TP IC7.P1(-2:EMC_A[09]/P1.9) IC10.H1(A9)
ABUS10: A10.TP IC7.P2(-2:EMC_A[10]/P1.10) IC10.J7(A10)
ABUS11: A11.TP IC7.P3(-2:EMC_A[11]/P1.11) IC10.H2(A11)
ABUS12: A12.TP IC7.N4(-2:EMC_A[12]/P1.12) IC10.H3(A12)
ABUS13: A13.TP IC7.R1(-2:EMC_A[13]/P1.13) IC10.H8(BA0)
ABUS14: A14.TP IC7.R2(-2:EMC_A[14]/P1.14) IC10.H9(BA1)
CPU_DDR_DQS0: C75.1 R26.2 R82.2 R86.1
CPU_DDR_DQS1: C74.1 R31.2 R84.2 R87.1
DBUS0: 0.TP IC7.U4(-4:EMC_D[00]) IC10.A8(DQ0)
DBUS1: 1.TP IC7.R7(-4:EMC_D[01]) IC10.B7(DQ1)
DBUS2: 2.TP IC7.T5(-4:EMC_D[02]) IC10.B8(DQ2)
DBUS3: 3.TP IC7.U5(-4:EMC_D[03]) IC10.C7(DQ3)
DBUS4: 4.TP IC7.V3(-4:EMC_D[04]) IC10.C8(DQ4)
DBUS5: 5.TP IC7.V4(-4:EMC_D[05]) IC10.D7(DQ5)
DBUS6: 6.TP IC7.T6(-4:EMC_D[06]) IC10.D8(DQ6)
DBUS7: 7.TP IC7.R8(-4:EMC_D[07]) IC10.E7(DQ7)
DBUS8: 8.TP IC7.V5(-4:EMC_D[08]) IC10.E3(DQ8)
DBUS9: 9.TP IC7.U6(-4:EMC_D[09]) IC10.D2(DQ9)
DBUS10: 10.TP IC7.V6(-4:EMC_D[10]) IC10.D3(DQ10)
DBUS11: 11.TP IC7.T7(-4:EMC_D[11]) IC10.C2(DQ11)
DBUS12: 12.TP IC7.U7(-4:EMC_D[12]) IC10.C3(DQ12)
DBUS13: 13.TP IC7.V7(-4:EMC_D[13]) IC10.B2(DQ13)
DBUS14: 14.TP IC7.T8(-4:EMC_D[14]) IC10.B3(DQ14)
DBUS15: 15.TP IC7.U8(-4:EMC_D[15]) IC10.A2(DQ15)
DDR_CKE: IC10.G1(CKE) R89.2
DDR_CLK: IC10.G2(CK) R33.2
DDR_DSQ0: IC10.E8(LDQS) R38.2 R83.2
DDR_DSQ1: IC10.E2(UDQS) R39.2 R85.2
DQM0: IC10.F8(LDM) RN9.8
DQM1: IC10.F2(UDM) RN9.7
DYCS0: IC10.H7(!CS) RN10.5
EMC_CLK: IC7.T3(-3:EMC_CLK) R33.1
GND [med_pow]: C67.2 C68.2 C74.2 C75.2 C76.2 C78.2 C79.2 C80.2 C81.2 C82.2 C83.2 IC9.13(VSS1) IC9.36(VSS2) IC10.A1(VSS0) IC10.A3(VSSQ0) IC10.B9(VSSQ1) IC10.C1(VSSQ2) IC10.D9(VSSQ3) IC10.E1(VSSQ4) IC10.F1(VSS1) IC10.K1(VSS2) R81.1 SP21.TP SP22.TP SP23.TP SP24.TP SP25.TP SP26.TP ; also sheet 2,3,5,6
GPO19/!WP_NAND: R79.1 ; also sheet 2
N$37: R38.1 R86.2
N$40: R39.1 R87.2
N$58: IC7.G2(-5:FLASH_IO[05]) IC9.42(IO5)
N$59: IC7.G3(-5:FLASH_IO[06]) IC9.43(IO6)
N$60: IC7.H2(-5:FLASH_IO[00]) IC9.29(IO0)
N$61: IC7.H3(-5:FLASH_IO[01]) IC9.30(IO1)
N$62: IC7.F1(-5:FLASH_IO[02]) IC9.31(IO2)
N$63: IC7.E1(-5:FLASH_IO[03]) IC9.32(IO3)
N$64: IC7.H4(-5:FLASH_IO[04]) IC9.41(IO4)
N$65: IC7.E2(-5:FLASH_IO[07]) IC9.44(IO7)
N$66: IC7.D2(-5:FLASH_ALE) IC9.17(ALE)
N$67: IC7.E3(-5:FLASH_CE_N) IC9.9(!CE)
N$68: IC7.F2(-5:FLASH_WR_N) IC9.18(!WE)
N$69: IC7.C1(-5:FLASH_RD_N) IC9.8(!RE)
N$70: IC7.F3(-5:FLASH_CLE) IC9.16(CLE)
N$71: IC7.D1(-5:FLASH_RDY) IC9.7(R/!B) R58.1
N$72: IC9.19(!WP) R78.1 R79.2
N$110: IC7.V8(-4:EMC_D[16]/DDR_DQS0) R26.1
N$111: IC7.R9(-4:EMC_D[17]/DDR_DQS1) R31.1
N$114: IC7.T2(-3:EMC_RAS_N) RN10.1
N$115: R82.1 R83.1
N$116: R84.1 R85.1
N$117: IC7.R5(-3:EMC_CAS_N) RN10.3
N$118: IC7.R4(-3:EMC_WR_N) RN10.2
N$119: IC7.R3(-3:EMC_DQM[0]) RN9.1
N$120: IC7.P4(-3:EMC_DQM[1]) RN9.2
N$121: IC7.R6(-3:EMC_DYCS0_N) RN10.4
N$122: IC7.U3(-3:EMC_CKE0) R89.1
VDD_3V3: C67.1 C68.1 IC9.12(VCC1) IC9.37(VCC2) R58.2 R78.2 ; also sheet 2,3,5,6
VDD_EMC: C77.1 C78.1 C79.1 C80.1 C81.1 C82.1 C83.1 IC10.A7(VDDQ0) IC10.A9(VDD0) IC10.B1(VDDQ1) IC10.C9(VDDQ2) IC10.D1(VDDQ3) IC10.E9(VDDQ4) IC10.F9(VDD1) IC10.K9(VDD2) R80.2 ; also sheet 6
Unconnected: IC7.G1(-3:EMC_DYCS1_N) IC7.H1(-3:EMC_OE_N) IC7.J1(-2:EMC_A[20]/P1.20) IC7.J2(-2:EMC_A[21]/P1.21) IC7.J3(-2:EMC_A[22]/P1.22) IC7.J4(-2:EMC_A[23]/P1.23) IC7.K1(-2:EMC_A[19]/P1.19) IC7.K2(-2:EMC_A[18]/P1.18) IC7.K3(-2:EMC_A[16]/P1.16) IC7.K4(-2:EMC_A[17]/P1.17) IC7.L1(-2:EMC_A[15]/P1.15) IC7.L2(-3:EMC_CKE1) IC7.P5(-3:EMC_DQM[3]) IC7.P12(-3:EMC_BLS[3]) IC7.R10(-4:EMC_D[24]/P2.5) IC7.R11(-3:EMC_CS1_N) IC7.R12(-3:EMC_BLS[2]) IC7.T1(-3:EMC_DQM[2]) IC7.T4(-3:EMC_CLKIN) IC7.T9(-4:EMC_D[20]/P2.1) IC7.T10(-4:EMC_D[23]/P2.4) IC7.T11(-4:EMC_D[27]/P2.8) IC7.T12(-3:EMC_CS2_N) IC7.T13(-3:EMC_BLS[1]) IC7.U9(-4:EMC_D[19]/P2.0) IC7.U10(-4:EMC_D[22]/P2.3) IC7.U11(-4:EMC_D[26]/P2.7) IC7.U12(-4:EMC_D[30]/P2.11) IC7.U13(-3:EMC_CS0_N) IC7.U14(-3:EMC_BLS[0]) IC7.V10(-4:EMC_D[21]/P2.2) IC7.V11(-4:EMC_D[25]/P2.6) IC7.V12(-4:EMC_D[28]/P2.9) IC7.V13(-4:EMC_D[29]/P2.10) IC7.V14(-4:EMC_D[31]/P2.12) IC7.V15(-3:EMC_CS3_N) IC10.F3(NC) IC10.F7(DNU) RN9.3 RN9.4 RN9.5 RN9.6

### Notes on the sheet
- 512Mb (32Mx16bit) Mobile DDR SDRAM
- Temp range: -30 ... +85 C
- Clock skew errata
- FLASH NAND 1Gb (128Mx8bit)
- Extra long route between micro and DDR
- 0 ... 70 C: H27U1G8F2BTR-BC
- -40 .. +85 C: NAND01GW3B2CN6E
- R.Hendricksen
- Main
- Memory
- © NXP Semiconductors | V1.1

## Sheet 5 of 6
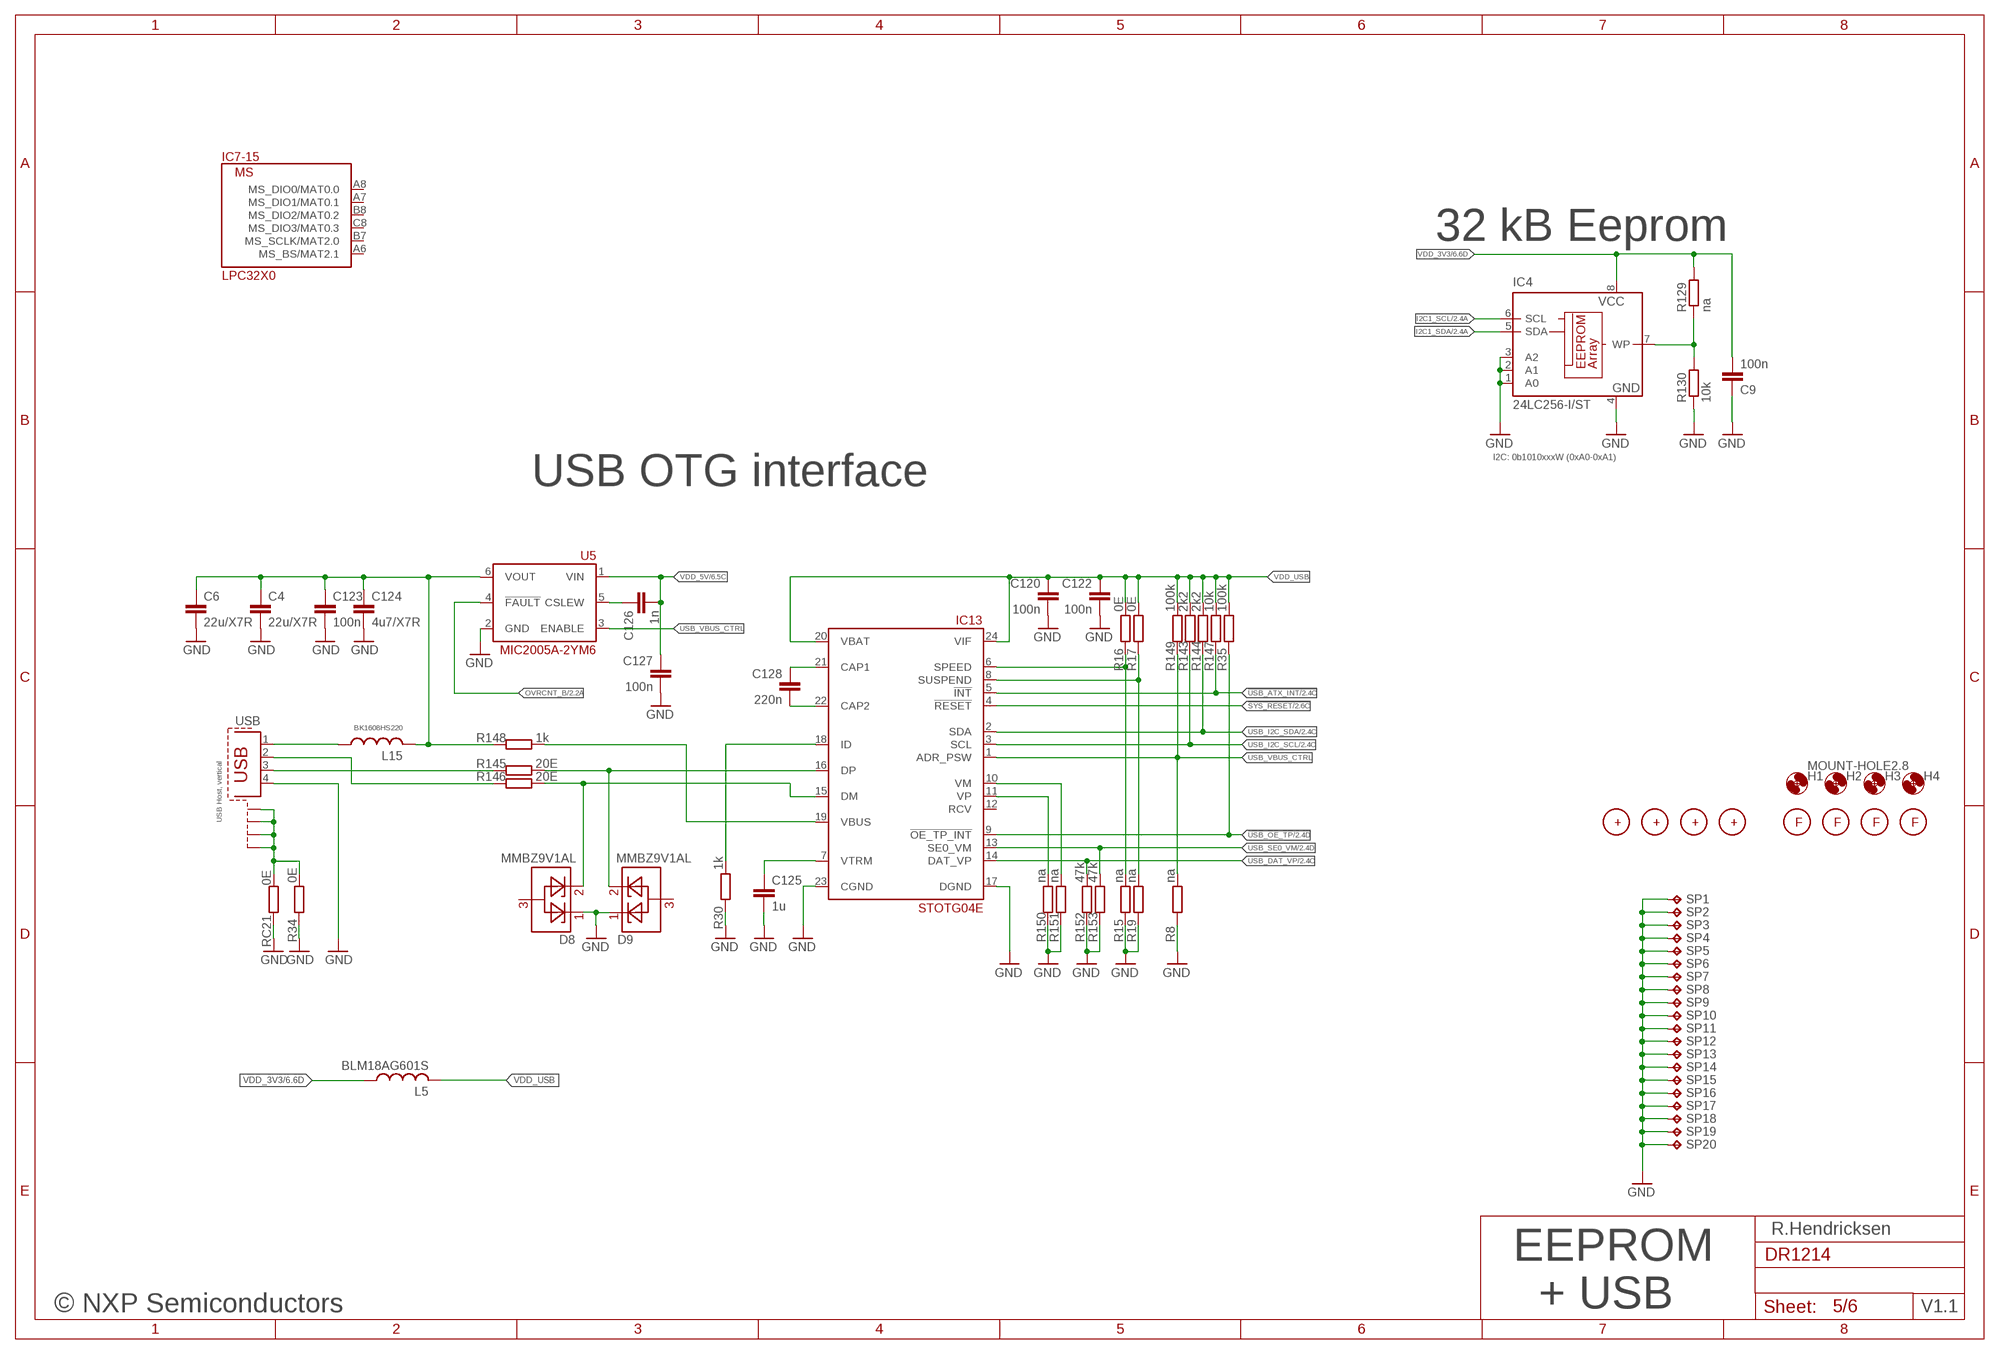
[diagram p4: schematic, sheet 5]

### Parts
C4  22u/X7R  C-EUC1206  [C1206]
C6  22u/X7R  C-EUC1206  [C1206]
C9  100n  C-EUC0402  [C0402]
C120  100n  C-EUC0402  [C0402]
C122  100n  C-EUC0402  [C0402]
C123  100n  C-EUC0402  [C0402]
C124  4u7/X7R  C-EUC0805  [C0805]
C125  1u  C-EUC0402  [C0402]
C126  1n  C-EUC0402  [C0402]
C127  100n  C-EUC0402  [C0402]
C128  220n  C-EUC0402  [C0402]
D8  MMBZ9V1AL  [SOT23]
D9  MMBZ9V1AL  [SOT23]
FM1  CROSSHAIR8MIL  [CROSSHAIR_8MIL]
FM2  CROSSHAIR8MIL  [CROSSHAIR_8MIL]
FM3  CROSSHAIR8MIL  [CROSSHAIR_8MIL]
FM4  CROSSHAIR8MIL  [CROSSHAIR_8MIL]
H1  MOUNT-HOLE2.8  [2,8]
H2  MOUNT-HOLE2.8  [2,8]
H3  MOUNT-HOLE2.8  [2,8]
H4  MOUNT-HOLE2.8  [2,8]
IC4  24LC256-I/ST  [TSSOP8]
IC13  STOTG04E  [HVQFN24-4X4]
L5  BLM18AG601S  [PACKAGE0603]
L15  BK1608HS220  L0603  [P0603]
R8  na  R-EU_R0402  [R0402]
R15  na  R-EU_R0402  [R0402]
R16  0E  R-EU_R0402  [R0402]
R17  0E  R-EU_R0402  [R0402]
R19  na  R-EU_R0402  [R0402]
R30  1k  R-EU_R0402  [R0402]
R34  0E  R-EU_R1206  [R1206]
R35  100k  R-EU_R0402  [R0402]
R129  na  R-EU_R0402  [R0402]
R130  10k  R-EU_R0402  [R0402]
R143  2k2  R-EU_R0402  [R0402]
R144  2k2  R-EU_R0402  [R0402]
R145  20E  R-EU_R0402  [R0402]
R146  20E  R-EU_R0402  [R0402]
R147  10k  R-EU_R0402  [R0402]
R148  1k  R-EU_R0402  [R0402]
R149  100k  R-EU_R0402  [R0402]
R150  na  R-EU_R0402  [R0402]
R151  na  R-EU_R0402  [R0402]
R152  47k  R-EU_R0402  [R0402]
R153  47k  R-EU_R0402  [R0402]
RC21  0E  R-EU_R1206  [R1206]
SP1  TPTP06SQ  [TP06SQ]
SP2  TPTP06SQ  [TP06SQ]
SP3  TPTP06SQ  [TP06SQ]
SP4  TPTP06SQ  [TP06SQ]
SP5  TPTP06SQ  [TP06SQ]
SP6  TPTP06SQ  [TP06SQ]
SP7  TPTP06SQ  [TP06SQ]
SP8  TPTP06SQ  [TP06SQ]
SP9  TPTP06SQ  [TP06SQ]
SP10  TPTP06SQ  [TP06SQ]
SP11  TPTP06SQ  [TP06SQ]
SP12  TPTP06SQ  [TP06SQ]
SP13  TPTP06SQ  [TP06SQ]
SP14  TPTP06SQ  [TP06SQ]
SP15  TPTP06SQ  [TP06SQ]
SP16  TPTP06SQ  [TP06SQ]
SP17  TPTP06SQ  [TP06SQ]
SP18  TPTP06SQ  [TP06SQ]
SP19  TPTP06SQ  [TP06SQ]
SP20  TPTP06SQ  [TP06SQ]
U5  MIC2005A-2YM6  [SOT23-6]
U$3  FICUDIAL_1MM-1  [FIDUCIAL_1MMCIRCLE]
U$4  FICUDIAL_1MM-1  [FIDUCIAL_1MMCIRCLE]
U$5  FICUDIAL_1MM-1  [FIDUCIAL_1MMCIRCLE]
U$6  FICUDIAL_1MM-1  [FIDUCIAL_1MMCIRCLE]
USB  USB_A_HU  [USB_A_HU]

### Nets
!SYS_RESET: IC13.4(!RESET) ; also sheet 2,3
!USB_ATX_INT: IC13.5(!INT) R147.1 ; also sheet 2
!USB_OE_TP: IC13.9(!OE_TP_INT) R35.1 ; also sheet 2
GND [med_pow]: C4.2 C6.2 C9.1 C120.2 C122.2 C123.2 C124.2 C125.2 C127.2 D8.1 D9.1 IC4.1(A0) IC4.2(A1) IC4.3(A2) IC4.4(GND) IC13.17(DGND) IC13.23(CGND) R8.1 R15.1 R19.1 R30.1 R34.1 R130.1 R150.1 R151.1 R152.1 R153.1 RC21.2 SP1.TP SP2.TP SP3.TP SP4.TP SP5.TP SP6.TP SP7.TP SP8.TP SP9.TP SP10.TP SP11.TP SP12.TP SP13.TP SP14.TP SP15.TP SP16.TP SP17.TP SP18.TP SP19.TP SP20.TP U5.2(GND) USB.4(GND) ; also sheet 2,3,4,6
I2C1_SCL: IC4.6(SCL) ; also sheet 2
I2C1_SDA: IC4.5(SDA) ; also sheet 2
N$7: L15.1 USB.1(VBUS)
N$8: IC13.19(VBUS) R148.2
N$10: IC13.18(ID) R30.2
N$11: IC13.6(SPEED) R15.2 R16.1
N$14: IC13.8(SUSPEND) R17.1 R19.2
N$156: IC4.7(WP) R129.1 R130.2
N$172: C4.1 C6.1 C123.1 C124.1 L15.2 R148.1 U5.6(VOUT)
N$177: R145.1 USB.3(D+)
N$178: R146.1 USB.2(D-)
N$179: D9.2 IC13.16(DP) R145.2
N$180: D8.2 IC13.15(DM) R146.2
N$182: C128.1 IC13.21(CAP1)
N$183: C125.1 IC13.7(VTRM)
N$184: C128.2 IC13.22(CAP2)
N$186: C126.1 U5.5(CSLEW)
N$187: IC13.11(VP) R150.2
N$188: IC13.10(VM) R151.2
OVRCNT_B: U5.4(!FAULT) ; also sheet 2
USB_DAT_VP: IC13.14(DAT_VP) R152.2 ; also sheet 2
USB_I2C_SCL: IC13.3(SCL) R143.1 ; also sheet 2
USB_I2C_SDA: IC13.2(SDA) R144.1 ; also sheet 2
USB_SE0_VM: IC13.13(SE0_VM) R153.2 ; also sheet 2
USB_SHIELD: R34.2 RC21.1 USB.P$5(S1) USB.P$6(S2) USB.P$7(S3) USB.P$8(S4)
USB_VBUS_CTRL: IC13.1(ADR_PSW) R8.2 R149.1 U5.3(ENABLE)
VDD_3V3: C9.2 IC4.8(VCC) L5.1 R129.2 ; also sheet 2,3,4,6
VDD_5V: C126.2 C127.1 U5.1(VIN) ; also sheet 2,6
VDD_USB: C120.1 C122.1 IC13.20(VBAT) IC13.24(VIF) L5.2 R16.2 R17.2 R35.2 R143.2 R144.2 R147.2 R149.2
Unconnected: D8.3 D9.3 IC7.A6(-15:MS_BS/MAT2.1) IC7.A7(-15:MS_DIO1/MAT0.1) IC7.A8(-15:MS_DIO0/MAT0.0) IC7.B7(-15:MS_SCLK/MAT2.0) IC7.B8(-15:MS_DIO2/MAT0.2) IC7.C8(-15:MS_DIO3/MAT0.3) IC13.12(RCV)

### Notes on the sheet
- 32 kB Eeprom
- I2C: 0b1010xxxW (0xA0-0xA1)
- USB OTG interface
- USB Host, vertical
- R.Hendricksen
- EEPROM
- © NXP Semiconductors | + USB | V1.1

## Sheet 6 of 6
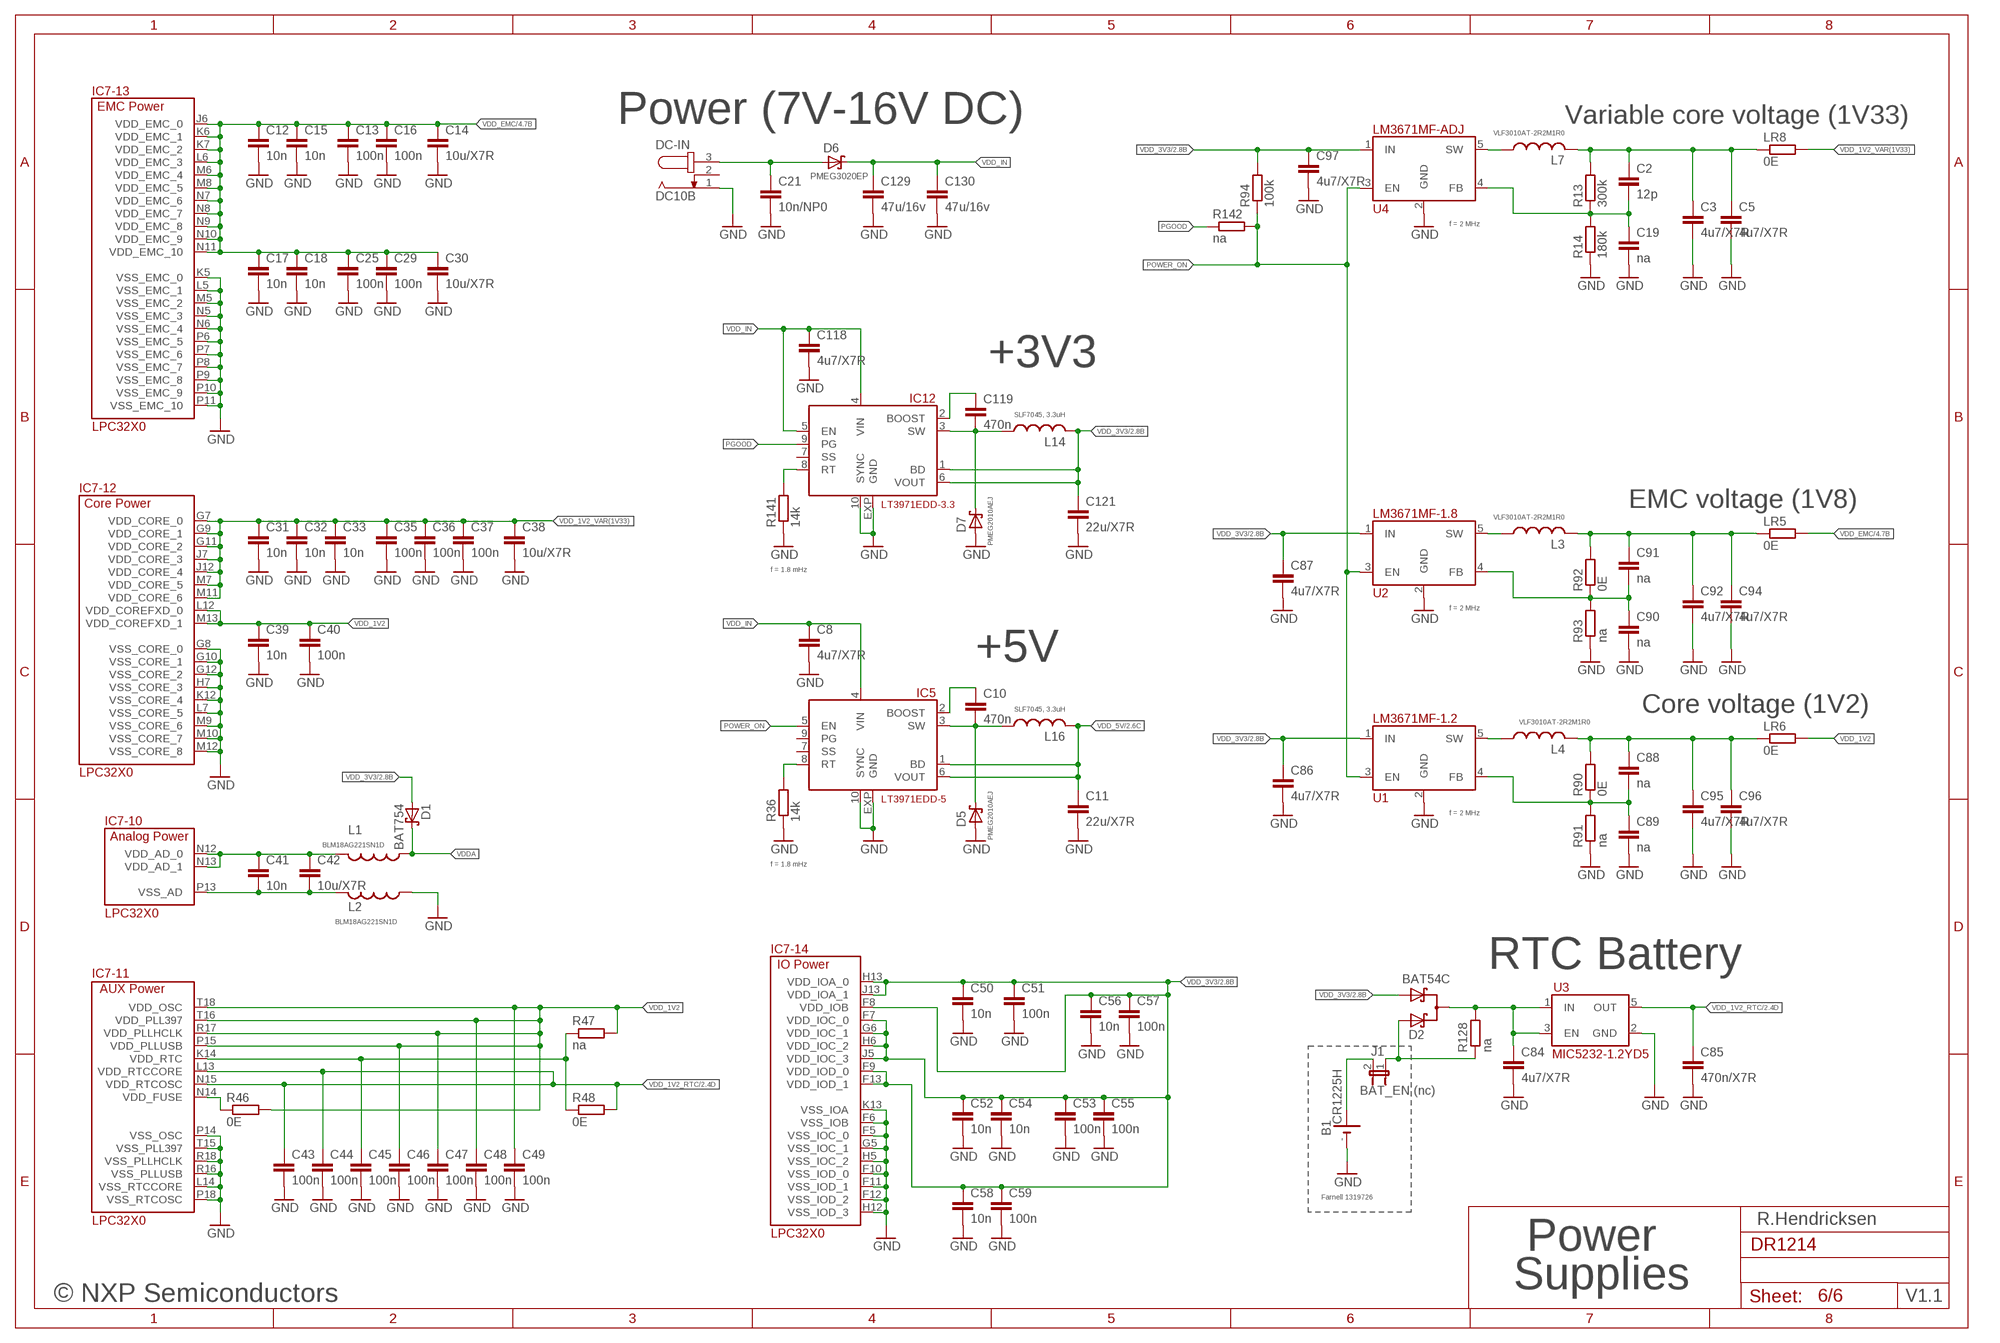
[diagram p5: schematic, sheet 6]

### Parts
B1  CR1225H  [CR1225H]
C2  12p  C-EUC0402  [C0402]
C3  4u7/X7R  C-EUC0805  [C0805]
C5  4u7/X7R  C-EUC0805  [C0805]
C8  4u7/X7R  C-EUC0805  [C0805]
C10  470n  C-EUC0603  [C0603]
C11  22u/X7R  C-EUC1206  [C1206]
C12  10n  C-EUC0402  [C0402]
C13  100n  C-EUC0402  [C0402]
C14  10u/X7R  C-EUC0805  [C0805]
C15  10n  C-EUC0402  [C0402]
C16  100n  C-EUC0402  [C0402]
C17  10n  C-EUC0402  [C0402]
C18  10n  C-EUC0402  [C0402]
C19  na  C-EUC0402  [C0402]
C21  10n/NP0  C-EUC0603  [C0603]
C25  100n  C-EUC0402  [C0402]
C29  100n  C-EUC0402  [C0402]
C30  10u/X7R  C-EUC0805  [C0805]
C31  10n  C-EUC0402  [C0402]
C32  10n  C-EUC0402  [C0402]
C33  10n  C-EUC0402  [C0402]
C35  100n  C-EUC0402  [C0402]
C36  100n  C-EUC0402  [C0402]
C37  100n  C-EUC0402  [C0402]
C38  10u/X7R  C-EUC0805  [C0805]
C39  10n  C-EUC0402  [C0402]
C40  100n  C-EUC0402  [C0402]
C41  10n  C-EUC0402  [C0402]
C42  10u/X7R  C-EUC0805  [C0805]
C43  100n  C-EUC0402  [C0402]
C44  100n  C-EUC0402  [C0402]
C45  100n  C-EUC0402  [C0402]
C46  100n  C-EUC0402  [C0402]
C47  100n  C-EUC0402  [C0402]
C48  100n  C-EUC0402  [C0402]
C49  100n  C-EUC0402  [C0402]
C50  10n  C-EUC0402  [C0402]
C51  100n  C-EUC0402  [C0402]
C52  10n  C-EUC0402  [C0402]
C53  100n  C-EUC0402  [C0402]
C54  10n  C-EUC0402  [C0402]
C55  100n  C-EUC0402  [C0402]
C56  10n  C-EUC0402  [C0402]
C57  100n  C-EUC0402  [C0402]
C58  10n  C-EUC0402  [C0402]
C59  100n  C-EUC0402  [C0402]
C84  4u7/X7R  C-EUC0805  [C0805]
C85  470n/X7R  C-EUC0603  [C0603]
C86  4u7/X7R  C-EUC0805  [C0805]
C87  4u7/X7R  C-EUC0805  [C0805]
C88  na  C-EUC0402  [C0402]
C89  na  C-EUC0402  [C0402]
C90  na  C-EUC0402  [C0402]
C91  na  C-EUC0402  [C0402]
C92  4u7/X7R  C-EUC0805  [C0805]
C94  4u7/X7R  C-EUC0805  [C0805]
C95  4u7/X7R  C-EUC0805  [C0805]
C96  4u7/X7R  C-EUC0805  [C0805]
C97  4u7/X7R  C-EUC0805  [C0805]
C118  4u7/X7R  C-EUC0805  [C0805]
C119  470n  C-EUC0603  [C0603]
C121  22u/X7R  C-EUC1206  [C1206]
C129  47u/16v  C-EUC1210  [C1210]
C130  47u/16v  C-EUC1210  [C1210]
D1  BAT754  BAS16  [SOT23]
D2  BAT54C  [SOT23]
D5  PMEG2010AEJ  [SOD323-W]
D6  PMEG3020EP  DIODE-SHOTTKY-SOD128  [SOD128]
D7  PMEG2010AEJ  [SOD323-W]
DC-IN  DC10B  JACK-PLUGBIGHOLES  [DC_BIGHOLES]
IC5  LT3971EDD-5  LT3971EDD-3.3  [DFN10-3X3]
IC12  LT3971EDD-3.3  [DFN10-3X3]
J1  BAT_EN (nc)  JP1E  [JP1]
L1  BLM18AG221SN1D  L_0603  [R0603]
L2  BLM18AG221SN1D  L_0603  [R0603]
L3  VLF3010AT-2R2M1R0  COIL2.8MM  [COIL2.8MM]
L4  VLF3010AT-2R2M1R0  COIL2.8MM  [COIL2.8MM]
L7  VLF3010AT-2R2M1R0  COIL2.8MM  [COIL2.8MM]
L14  SLF7045, 3.3uH  COIL70X70  [COIL7070]
L16  SLF7045, 3.3uH  COIL70X70  [COIL7070]
LR5  0E  R-EU_R0603  [R0603]
LR6  0E  R-EU_R0603  [R0603]
LR8  0E  R-EU_R0603  [R0603]
R13  300k  R-EU_R0402  [R0402]
R14  180k  R-EU_R0402  [R0402]
R36  14k  R-EU_R0402  [R0402]
R46  0E  R-EU_R0402  [R0402]
R47  na  R-EU_R0402  [R0402]
R48  0E  R-EU_R0402  [R0402]
R90  0E  R-EU_R0402  [R0402]
R91  na  R-EU_R0402  [R0402]
R92  0E  R-EU_R0402  [R0402]
R93  na  R-EU_R0402  [R0402]
R94  100k  R-EU_R0402  [R0402]
R128  na  R-EU_R0402  [R0402]
R141  14k  R-EU_R0402  [R0402]
R142  na  R-EU_R0402  [R0402]
U1  LM3671MF-1.2  [SOT23-5]
U2  LM3671MF-1.8  [SOT23-5]
U3  MIC5232-1.2YD5  MIC5232-1.2YD2  [SOT23-5]
U4  LM3671MF-ADJ  LM3671MF-1.8  [SOT23-5]

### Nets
GND [med_pow]: B1.- C3.2 C5.2 C8.2 C11.2 C12.2 C13.2 C14.2 C15.2 C16.2 C17.2 C18.2 C19.2 C21.2 C25.2 C29.2 C30.2 C31.2 C32.2 C33.2 C35.2 C36.2 C37.2 C38.2 C39.2 C40.2 C43.2 C44.2 C45.2 C46.2 C47.2 C48.2 C49.2 C50.2 C51.2 C52.2 C53.2 C54.2 C55.2 C56.2 C57.2 C58.2 C59.2 C84.2 C85.2 C86.2 C87.2 C89.2 C90.2 C92.2 C94.2 C95.2 C96.2 C97.2 C118.2 C121.2 C129.2 C130.2 D5.A D7.A DC-IN.1 IC5.10(SYNC) IC5.EXP(GND) IC7.F5(-14:VSS_IOC_0) IC7.F6(-14:VSS_IOB) IC7.F10(-14:VSS_IOD_0) IC7.F11(-14:VSS_IOD_1) IC7.F12(-14:VSS_IOD_2) IC7.G5(-14:VSS_IOC_1) IC7.G8(-12:VSS_CORE_0) IC7.G10(-12:VSS_CORE_1) IC7.G12(-12:VSS_CORE_2) IC7.H5(-14:VSS_IOC_2) IC7.H7(-12:VSS_CORE_3) IC7.H12(-14:VSS_IOD_3) IC7.K5(-13:VSS_EMC_0) IC7.K12(-12:VSS_CORE_4) IC7.K13(-14:VSS_IOA) IC7.L5(-13:VSS_EMC_1) IC7.L7(-12:VSS_CORE_5) IC7.L14(-11:VSS_RTCCORE) IC7.M5(-13:VSS_EMC_2) IC7.M9(-12:VSS_CORE_6) IC7.M10(-12:VSS_CORE_7) IC7.M12(-12:VSS_CORE_8) IC7.N5(-13:VSS_EMC_3) IC7.N6(-13:VSS_EMC_4) IC7.P6(-13:VSS_EMC_5) IC7.P7(-13:VSS_EMC_6) IC7.P8(-13:VSS_EMC_7) IC7.P9(-13:VSS_EMC_8) IC7.P10(-13:VSS_EMC_9) IC7.P11(-13:VSS_EMC_10) IC7.P14(-11:VSS_OSC) IC7.P18(-11:VSS_RTCOSC) IC7.R16(-11:VSS_PLLUSB) IC7.R18(-11:VSS_PLLHCLK) IC7.T15(-11:VSS_PLL397) IC12.10(SYNC) IC12.EXP(GND) L2.1 R14.1 R36.1 R91.1 R93.1 R141.1 U1.2(GND) U2.2(GND) U3.2(GND) U4.2(GND) ; also sheet 2,3,4,5
N$9: C41.1 C42.1 IC7.N12(-10:VDD_AD_0) IC7.N13(-10:VDD_AD_1) L1.2
N$13: IC5.8(RT) R36.2
N$16: C10.1 IC5.2(BOOST)
N$17: C21.1 D6.A DC-IN.3
N$21: C41.2 C42.2 IC7.P13(-10:VSS_AD) L2.2
N$22: IC7.N14(-11:VDD_FUSE) R46.1
N$24: C45.1 IC7.K14(-11:VDD_RTC) R47.1 R48.1
N$27: C2.2 C19.1 R13.1 R14.2 U4.4(FB)
N$28: L7.P$1 U4.5(SW)
N$29: C2.1 C3.1 C5.1 L7.P$2 LR8.1 R13.2
N$123: C84.1 D2.3(CC) R128.2 U3.1(IN) U3.3(EN)
N$127: C88.2 C89.1 R90.1 R91.2 U1.4(FB)
N$128: C90.1 C91.2 R92.1 R93.2 U2.4(FB)
N$129: L4.P$1 U1.5(SW)
N$130: C88.1 C95.1 C96.1 L4.P$2 LR6.1 R90.2
N$131: L3.P$1 U2.5(SW)
N$132: C91.1 C92.1 C94.1 L3.P$2 LR5.1 R92.2
N$154 [med_pow]: B1.+ J1.2
N$155 [med_pow]: D2.1(A1) J1.1 R128.1
N$173: IC12.8(RT) R141.2
N$175: C119.1 IC12.2(BOOST)
PGOOD: IC12.9(PG) R142.1
POWER_ON: IC5.5(EN) R94.1 R142.2 U1.3(EN) U2.3(EN) U4.3(EN)
SW_3V3: C119.2 D7.C IC12.3(SW) L14.1
SW_5V: C10.2 D5.C IC5.3(SW) L16.1
VDD_1V2: C39.1 C40.1 C46.1 C47.1 C48.1 C49.1 IC7.L12(-12:VDD_COREFXD_0) IC7.M13(-12:VDD_COREFXD_1) IC7.P15(-11:VDD_PLLUSB) IC7.R17(-11:VDD_PLLHCLK) IC7.T16(-11:VDD_PLL397) IC7.T18(-11:VDD_OSC) LR6.2 R46.2 R47.2
VDD_1V2_RTC: C43.1 C44.1 C85.1 IC7.L13(-11:VDD_RTCCORE) IC7.N15(-11:VDD_RTCOSC) R48.2 U3.5(OUT) ; also sheet 2
VDD_1V2_VAR(1V33): C31.1 C32.1 C33.1 C35.1 C36.1 C37.1 C38.1 IC7.G7(-12:VDD_CORE_0) IC7.G9(-12:VDD_CORE_1) IC7.G11(-12:VDD_CORE_2) IC7.J7(-12:VDD_CORE_3) IC7.J12(-12:VDD_CORE_4) IC7.M7(-12:VDD_CORE_5) IC7.M11(-12:VDD_CORE_6) LR8.2
VDD_3V3: C50.1 C51.1 C52.1 C53.1 C54.1 C55.1 C56.1 C57.1 C58.1 C59.1 C86.1 C87.1 C97.1 C121.1 D1.1(A) D2.2(A2) IC7.F7(-14:VDD_IOC_0) IC7.F8(-14:VDD_IOB) IC7.F9(-14:VDD_IOD_0) IC7.F13(-14:VDD_IOD_1) IC7.G6(-14:VDD_IOC_1) IC7.H6(-14:VDD_IOC_2) IC7.H13(-14:VDD_IOA_0) IC7.J5(-14:VDD_IOC_3) IC7.J13(-14:VDD_IOA_1) IC12.1(BD) IC12.6(VOUT) L14.2 R94.2 U1.1(IN) U2.1(IN) U4.1(IN) ; also sheet 2,3,4,5
VDD_5V: C11.1 IC5.1(BD) IC5.6(VOUT) L16.2 ; also sheet 2,5
VDD_EMC: C12.1 C13.1 C14.1 C15.1 C16.1 C17.1 C18.1 C25.1 C29.1 C30.1 IC7.J6(-13:VDD_EMC_0) IC7.K6(-13:VDD_EMC_1) IC7.K7(-13:VDD_EMC_2) IC7.L6(-13:VDD_EMC_3) IC7.M6(-13:VDD_EMC_4) IC7.M8(-13:VDD_EMC_5) IC7.N7(-13:VDD_EMC_6) IC7.N8(-13:VDD_EMC_7) IC7.N9(-13:VDD_EMC_8) IC7.N10(-13:VDD_EMC_9) IC7.N11(-13:VDD_EMC_10) LR5.2 ; also sheet 4
VDD_IN: C8.1 C118.1 C129.1 C130.1 D6.C IC5.4(VIN) IC12.4(VIN) IC12.5(EN)
VDDA: D1.3(C) L1.1
Unconnected: DC-IN.2 IC5.7(SS) IC5.9(PG) IC12.7(SS)

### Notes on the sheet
- Power (7V-16V DC) | Variable core voltage (1V33)
- f = 2 MHz
- +3V3
- EMC voltage (1V8)
- f = 1.8 mHz
- f = 2 MHz
- +5V
- Core voltage (1V2)
- f = 2 MHz
- f = 1.8 mHz
- RTC Battery
- Farnell 1319726
- R.Hendricksen
- Power
- Supplies
- © NXP Semiconductors | V1.1

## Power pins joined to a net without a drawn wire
GND: RF.3(GND) RF.4(GND) RF.5(GND)

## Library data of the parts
0 1-15 A0 A1-A14 = 11_rudhen_misc:TP
B1 = 11_rudhen:CR1225H: Battery
BUT1 BUT2 = rudhen:MCDTS
C1-C6 C8-C19 C21 C25 C26 C29-C92 C94-C97 C103-C106 C108-C132 C134-C141 = 11_rcl:C-EU: CAPACITOR, European symbol
C20 = 11_rcl:C-TRIMM: Trimm capacitor
C133 = RCL:C-EU: CAPACITOR, European symbol
D1 D3 D4 D10 D11 = 11_rudhen_diode:BAS16: Silicon Schottky Diodes
D2 = 11_rudhen_diode:BAT54C: Schottky Diodes Source: Fairchild .. BAT54.pdf
D5 D7 = 11_rudhen_diode:PMEG2010
D6 = 11_rudhen_diode:DIODE-SHOTTKY
D8 D9 = 11_rudhen_diode:MMBZ9V1AL: Low capacitance unidirectional double ESD protection diodes
DC-IN = 11_rudhen_con:JACK-PLUG: DC POWER JACK Power Jack, DC, Right Angle, Through Hole, Rated 5A at 16VDC, PC Terminals Distributor: Farnell (www.Farnell.de) Drawing: 84N1161.pdf / 84N1162.pdf Manufacturer: SPC Technology (www.spctechnology.com) Type: SPC4077 / SPC 4078
ETH = 11_rudhen:JACK8LED_RH
EXT = 11_rudhen_con:M50-3601042: Fabrikant: HARWIN, ordercode: 1022311, Fabrikantnummer: M50-3601042 HEADER, SMT, 2ROW, 20WAY Connector Type:Board to Board Pitch Spacing:1.27mm No. of Rows:2 No. of Contacts:20 Contact Termination:Surface Mount Vertical
FM1-FM4 = pickplace:CROSSHAIR: Crosshair fiducial mark
H1-H4 = holes:MOUNT-HOLE: MOUNTING HOLE with drill center marker
IC1 = 11_rudhen_power:CAT811S: 4-Pin Microprocessor Power Supply Supervisors with Manual Reset
IC2 IC8 = 74xx-little-de:74*1G125: Single Bus Buffer Gate with 3-State Output
IC4 = 11_rudhen_memory:24LC256
IC5 IC12 = 11_rudhen_power:LT3971: 38V, 1.2A, 2MHz Step-Down Regulator with 2.8?A Quiescent Current
IC7 = 11_rudhen_lpc32x0:LPC32X0
IC9 = 11_rudhen_memory:H27U1G8F2B
IC10 = 11_rudhen_memory:H5MS5162EFR
IC11 = 11_rudhen_lpc:JN516X
IC13 = 11_rudhen_misc:STOTG04E: USB-OTG Full-speed Transceiver
J1 = JUMPER:JP1E: JUMPER
J_TP1 J_TP2 SP1-SP26 TC1 TC2 = testpad:TP: Test pad
JTAG = 11_rudhen_con:M50: Samtec connector, 10-way
JUART1 = Non-NXP_60:BD075-06-A-1-L-D: GLOBAL CONNECTOR TECHNOLOGY - BD075-06-A-1-L-D - BOARD-BOARD CONNECTOR SOCKET, 6WAY, 1ROW
L1 L2 L11 = 11_rudhen_rcl:L_0603
L3 L4 L7 = 11_rudhen_rcl:COIL2.8MM: Coil radial, 2.8 mm
L5 L6 L8 L17 = rudhen:BLM18AG
L12 L13 L15 = 11_rcl:L: Inductor
L14 L16 = 11_rudhen_rcl:COIL70X70
LED1-LED6 = 11_rudhen_led_opto:OVS: Chip LED 0805
LR5 LR6 LR8 R1-R40 R46-R50 R52-R56 R58 R61-R65 R68 R71-R74 R78-R87 R89-R94 R105-R113 R128-R132 R135-R153 RC21 RC22 = 11_rcl:R-EU_: RESISTOR, European symbol
PROG = 11_rudhen_switch:B3: 6.2 X 6.5mm TACT Switch (SMD)
Q4 = rudhen:RTCCRYSTAL
Q5 Q12 = rudhen:CRYSTAL4
Q201 = MVer_Ethernet:ASEMPC-50.000MHZ-LR-T: PERFORMANCE PLASTIC PACKAGE ULTRA MINIATURE 3.2 x 2.5 x 0.85 mm PURE SILICONTM CLOCK OSCILLATOR Source: http://www.abracon.com/Oscillators/ASEMP.pdf; FARNELL: 1960717; OC_FARNELL: unknown; OC_NEWARK: unknown
RESET = 11_rudhen_switch:MCDTS: Tact switch, vertical, through-hole
RF = con-coax:BU-SMA-V: FEMALE SMA CONNECTOR Radiall distributor RS 112-3794; OC_FARNELL: unknown; OC_NEWARK: unknown
RN9 RN10 = resistor-dil:4R-N: Array Chip Resistor Source: RS Component / Phycomp; OC_FARNELL: unknown; OC_NEWARK: unknown
U1 U2 U4 = 11_rudhen_power:LM3671: LM3671MF-1.2/NOPB - IC, DC DC CONVERTER
U3 = 11_rudhen_power:MIC5232: MIC5232-1.2YD5 TR - LDO, 0.1VDO, 0.01A, 1.2V, 3%, 5TSOT23
U5 = 11_rudhen_transistor:MIC2005: Fixed Current Limit Power Distribution Switch with kickstart and slew rate control
U201 = 11_rudhen_misc:DP83848-2: DP83848 (40-LLP) - Single Port 10/100 Ethernet Transceiver Digikey: DP83848JSQCT-ND
U$1 = 11_rudhen_led_opto:LIGHTPIPE6
U$3-U$6 = pickplace:FICUDIAL_1MM
UART5 = pinhead-2:PINHD-1X06: PIN HEADER
USB = 11_rudhen_con:USB_A_HU

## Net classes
1 high_pow: width 1.27 mm
2 med_pow: width 0.61 mm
